(* Logix 5000 AddOnInstructionDefinition export AOI_NTron_7026TX_v1_2; software revision 20.04 *)

TYPE UDT_NTRON_Switch_Common_v1 :   // Created to use UDT_NTRON_CIP_Switch_v1
STRUCT
   Generic_Inputs : UDT_NTRON_Switch_In_v0;   // assembly received from switch
   Output : DINT;   // assembly sent to switch
   Identity : UDT_NTRON_CIP_Identity_v0;
   TCPIP : UDT_NTRON_CIP_TCPIP_Interface_v0;
   Switch : UDT_NTRON_CIP_Switch_v1;
   Ethernet_Link : UDT_NTRON_CIP_Ethernet_Link_v0[64];
   Data : UDT_NTRON_CIP_DATA_v0;   // Related to HMI data and control
   Control : UDT_NTRON_CIP_Control_v0;
END_STRUCT
END_TYPE

TYPE UDT_NTRON_CIP_Interface_Control_v0 :
STRUCT
   Control_Bits : INT;
   Forced_Interface_Speed : INT;
END_STRUCT
END_TYPE

TYPE UDT_NTRON_Switch_7026TX_In_v0 :   // N-TRON 7026TX Switch 26 Port (24 10/100BaseTX, 2 SFP Mini-GBIC Gigabit Fiber Expansion Ports)
STRUCT
   System_Faults : UDT_NTRON_System_Faults_v0;
   Admin_Status : DINT;   // AdminStatus of first 32 ports
   Admin_Status_P1 : BOOL;   // 1=enabled, 0=disabled
   Admin_Status_P2 : BOOL;
   Admin_Status_P3 : BOOL;
   Admin_Status_P4 : BOOL;
   Admin_Status_P5 : BOOL;
   Admin_Status_P6 : BOOL;
   Admin_Status_P7 : BOOL;
   Admin_Status_P8 : BOOL;
   Admin_Status_P9 : BOOL;
   Admin_Status_P10 : BOOL;
   Admin_Status_P11 : BOOL;
   Admin_Status_P12 : BOOL;
   Admin_Status_P13 : BOOL;
   Admin_Status_P14 : BOOL;
   Admin_Status_P15 : BOOL;
   Admin_Status_P16 : BOOL;
   Admin_Status_P17 : BOOL;
   Admin_Status_P18 : BOOL;
   Admin_Status_P19 : BOOL;
   Admin_Status_P20 : BOOL;
   Admin_Status_P21 : BOOL;
   Admin_Status_P22 : BOOL;
   Admin_Status_P23 : BOOL;
   Admin_Status_P24 : BOOL;
   Admin_Status_P25 : BOOL;
   Admin_Status_P26 : BOOL;
   Link_Status : DINT;   // LinkStatus of first 32 ports
   Link_Status_P1 : BOOL;   // 1=active, 0=inactive
   Link_Status_P2 : BOOL;
   Link_Status_P3 : BOOL;
   Link_Status_P4 : BOOL;
   Link_Status_P5 : BOOL;
   Link_Status_P6 : BOOL;
   Link_Status_P7 : BOOL;
   Link_Status_P8 : BOOL;
   Link_Status_P9 : BOOL;
   Link_Status_P10 : BOOL;
   Link_Status_P11 : BOOL;
   Link_Status_P12 : BOOL;
   Link_Status_P13 : BOOL;
   Link_Status_P14 : BOOL;
   Link_Status_P15 : BOOL;
   Link_Status_P16 : BOOL;
   Link_Status_P17 : BOOL;
   Link_Status_P18 : BOOL;
   Link_Status_P19 : BOOL;
   Link_Status_P20 : BOOL;
   Link_Status_P21 : BOOL;
   Link_Status_P22 : BOOL;
   Link_Status_P23 : BOOL;
   Link_Status_P24 : BOOL;
   Link_Status_P25 : BOOL;
   Link_Status_P26 : BOOL;
   Utilization_Alarm : DINT;   // Bandwith utilization alarms for first 32 ports
   Utilization_Alarm_P1 : BOOL;
   Utilization_Alarm_P2 : BOOL;
   Utilization_Alarm_P3 : BOOL;
   Utilization_Alarm_P4 : BOOL;
   Utilization_Alarm_P5 : BOOL;
   Utilization_Alarm_P6 : BOOL;
   Utilization_Alarm_P7 : BOOL;
   Utilization_Alarm_P8 : BOOL;
   Utilization_Alarm_P9 : BOOL;
   Utilization_Alarm_P10 : BOOL;
   Utilization_Alarm_P11 : BOOL;
   Utilization_Alarm_P12 : BOOL;
   Utilization_Alarm_P13 : BOOL;
   Utilization_Alarm_P14 : BOOL;
   Utilization_Alarm_P15 : BOOL;
   Utilization_Alarm_P16 : BOOL;
   Utilization_Alarm_P17 : BOOL;
   Utilization_Alarm_P18 : BOOL;
   Utilization_Alarm_P19 : BOOL;
   Utilization_Alarm_P20 : BOOL;
   Utilization_Alarm_P21 : BOOL;
   Utilization_Alarm_P22 : BOOL;
   Utilization_Alarm_P23 : BOOL;
   Utilization_Alarm_P24 : BOOL;
   Utilization_Alarm_P25 : BOOL;
   Utilization_Alarm_P26 : BOOL;
   Class1_Connections : INT;   // Number of CIP Ethernet/IP class 1 (multicast) connections
   Class3_Connections : INT;   // Number of CIP Ethernet/IP class 3 (unicast) connections
   Temperature_C : INT;   // Temperature in degrees Celsius. 0x7FFF = Not supported on device.
   Temperature_F : INT;   // Temperature in degrees Fahrenheit. 0x7FFF = Not supported on device.
   CPU_Utilization : SINT;   // Percent of CPU usage, 0-100
   Contact_Status : SINT;   // 2 Bits per contact. 00=Not Present, 01=Open, 10=Closed.
   Utilization_P1 : SINT;
   Utilization_P2 : SINT;
   Utilization_P3 : SINT;
   Utilization_P4 : SINT;
   Utilization_P5 : SINT;
   Utilization_P6 : SINT;
   Utilization_P7 : SINT;
   Utilization_P8 : SINT;
   Utilization_P9 : SINT;
   Utilization_P10 : SINT;
   Utilization_P11 : SINT;
   Utilization_P12 : SINT;
   Utilization_P13 : SINT;
   Utilization_P14 : SINT;
   Utilization_P15 : SINT;
   Utilization_P16 : SINT;
   Utilization_P17 : SINT;
   Utilization_P18 : SINT;
   Utilization_P19 : SINT;
   Utilization_P20 : SINT;
   Utilization_P21 : SINT;
   Utilization_P22 : SINT;
   Utilization_P23 : SINT;
   Utilization_P24 : SINT;
   Utilization_P25 : SINT;
   Utilization_P26 : SINT;
END_STRUCT
END_TYPE

TYPE UDT_NTRON_CIP_DATA_v0 :   // This UDT contains various information that appears on an HMI display. Some information applies to the switch, and some applies to the selected port (copied, or derived from, the port Ethernet_Link data) because FactoryTalk can not access array elements.
STRUCT
   Switch_Name : STRING;
   IP_Address : UDT_NTRON_String32;
   Subnet_Mask : UDT_NTRON_String32;
   Gateway_Address : UDT_NTRON_String32;
   Port_Speed : DINT;   // begin port specific data
   Port_Interface_Flags : UDT_NTRON_CIP_Interface_Flags_v0;
   Port_Interface_Label : STRING;
   Port_Interface_Type : SINT;   // 0-unknown, 1-internal, 2-twisted pair, 3-optical
   InOctets : DINT;
   InUcastPackets : DINT;
   InNucastPackets : DINT;
   OutOctets : DINT;
   OutUcastPackets : DINT;
   OutNucastPackets : DINT;
   Port : SINT;   // end port specific data
   MAC_Address : UDT_NTRON_String32;   // MAC address of switch
   TX_Unicast_Packet_Rate : DINT;   // begin port specific data
   RX_Unicast_Packet_Rate : DINT;
   TX_Multicast_Packet_Rate : DINT;
   RX_Multicast_Packet_Rate : DINT;
   TX_Broadcast_Packet_Rate : DINT;
   RX_Broadcast_Packet_Rate : DINT;
   Interface_Utilization : SINT;
   Port_Role : DINT;
   Error_Count : DINT;
   Fault_Count : DINT;   // end port specific data
   AOI_Major_Version : DINT;   // The faceplate reads this version to determine if the AOI tags can be used by the faceplate. If not, a warning is displayed.
   AOI_Minor_Version : DINT;   // The faceplate reads this version to determine if the AOI tags can be used by the faceplate. If not, a warning is displayed.
   CIP_Version_Fault : BOOL;   // True if the switch CIP version does not support this version of the AOI, otherwise false.
   Stale_Data : BOOL;   // True if assembly data has not been received lately.
   System_Fault_String : UDT_NTRON_String480;
END_STRUCT
END_TYPE

TYPE UDT_NTRON_CIP_Interface_Flags_v0 :
STRUCT
   Link_Status : BOOL;   // 0-inactive, 1-active
   Duplex : BOOL;   // 0-half, 1-full
   Negotiation_Status_1 : BOOL;
   Negotiation_Status_2 : BOOL;
   Negotiation_Status_3 : BOOL;
   Manual_Setting_Requires_Reset : BOOL;
   Local_Hardware_Fault : BOOL;
END_STRUCT
END_TYPE

TYPE UDT_NTRON_CIP_Control_v0 :   // Created to control explicit CIP messaging
STRUCT
   HMI : UDT_NTRON_HMI_Control_v0[1];   // Read Ethernet Link object for the selected port. 0=disabled.
   Selected_Port : INT;   // Use this member to read Ethernet Link object for one port. To read more than one port, use Read_Port_Mask. Set by the faceplate. Port data is copied to the UDT_NTRON_CIP_DATA_v0 data type.
   Request_Data : BOOL;   // 0 - explicit messaging is disabled; 1 - explicit messaging is enabled
   Read_Port_Mask : DINT;   // Set bit n to read ethernet link object for port n+1
   Read_Port_Mask2 : DINT;   // Set bit n to read ethernet link object for port n+33
   Explicit_Messaging_Timer_Reset : DINT;   // Used to control time between each MSG call to read CIP Identity object, TCPIP object, N-TRON object, and selected Ethernet Link objects. Minimum is 200 ms. Default is 1000 ms.
END_STRUCT
END_TYPE

TYPE UDT_NTRON_CIP_TCPIP_Interface_v0 :   // N-TRON CIP TCP/IP Interface Object
STRUCT
   Status : DINT;   // Interface status
   Configuration_Capability : DINT;   // Interface capability flags
   Configuration_Control : DINT;   // Interface control flags
   Path_Size : INT;   // Size of Path
   Object_Path_1 : INT;   // Logical segments identifying the physical link object
   Object_Path_2 : INT;   // Logical segments identifying the physical link object
   IP_Address : DINT;   // The device’s IP address.
   Network_Mask : DINT;   // The device’s network mask
   Gateway_Address : DINT;   // Default gateway address
   Name_Server_1 : DINT;   // Primary name server
   Name_Server_2 : DINT;   // Secondary name server
   Domain_Name : STRING;   // Default domain name
   Host_Name : STRING;   // Host name
END_STRUCT
END_TYPE

TYPE UDT_NTRON_Switch_In_v0 :   // Generic view of assembly data received from an N-TRON Switch. This UDT must match exactly the assembly sent from the switch.
STRUCT
   System_Faults : UDT_NTRON_System_Faults_v0;   // Status of various system faults.
   Admin_Status : DINT;   // Admin_Status of first 32 ports. Also available as port specific tags.
   Admin_Status_1 : BOOL;   // 1=enabled, 0=disabled
   Admin_Status_2 : BOOL;
   Admin_Status_3 : BOOL;
   Admin_Status_4 : BOOL;
   Admin_Status_5 : BOOL;
   Admin_Status_6 : BOOL;
   Admin_Status_7 : BOOL;
   Admin_Status_8 : BOOL;
   Admin_Status_9 : BOOL;
   Admin_Status_10 : BOOL;
   Admin_Status_11 : BOOL;
   Admin_Status_12 : BOOL;
   Admin_Status_13 : BOOL;
   Admin_Status_14 : BOOL;
   Admin_Status_15 : BOOL;
   Admin_Status_16 : BOOL;
   Admin_Status_17 : BOOL;
   Admin_Status_18 : BOOL;
   Admin_Status_19 : BOOL;
   Admin_Status_20 : BOOL;
   Admin_Status_21 : BOOL;
   Admin_Status_22 : BOOL;
   Admin_Status_23 : BOOL;
   Admin_Status_24 : BOOL;
   Admin_Status_25 : BOOL;
   Admin_Status_26 : BOOL;
   Admin_Status_27 : BOOL;
   Admin_Status_28 : BOOL;
   Admin_Status_29 : BOOL;
   Admin_Status_30 : BOOL;
   Admin_Status_31 : BOOL;
   Admin_Status_32 : BOOL;
   Admin_Status2 : DINT;   // Admin_Status of second 32 ports. Also available as port specific tags.
   Admin_Status_33 : BOOL;   // 1=enabled, 0=disabled
   Admin_Status_34 : BOOL;
   Admin_Status_35 : BOOL;
   Admin_Status_36 : BOOL;
   Admin_Status_37 : BOOL;
   Admin_Status_38 : BOOL;
   Admin_Status_39 : BOOL;
   Admin_Status_40 : BOOL;
   Admin_Status_41 : BOOL;
   Admin_Status_42 : BOOL;
   Admin_Status_43 : BOOL;
   Admin_Status_44 : BOOL;
   Admin_Status_45 : BOOL;
   Admin_Status_46 : BOOL;
   Admin_Status_47 : BOOL;
   Admin_Status_48 : BOOL;
   Admin_Status_49 : BOOL;
   Admin_Status_50 : BOOL;
   Admin_Status_51 : BOOL;
   Admin_Status_52 : BOOL;
   Admin_Status_53 : BOOL;
   Admin_Status_54 : BOOL;
   Admin_Status_55 : BOOL;
   Admin_Status_56 : BOOL;
   Admin_Status_57 : BOOL;
   Admin_Status_58 : BOOL;
   Admin_Status_59 : BOOL;
   Admin_Status_60 : BOOL;
   Admin_Status_61 : BOOL;
   Admin_Status_62 : BOOL;
   Admin_Status_63 : BOOL;
   Admin_Status_64 : BOOL;
   Link_Status : DINT;   // Link_Status of first 32 ports. Also available as port specific tags.
   Link_Status_1 : BOOL;   // 1=active, 0=inactive
   Link_Status_2 : BOOL;
   Link_Status_3 : BOOL;
   Link_Status_4 : BOOL;
   Link_Status_5 : BOOL;
   Link_Status_6 : BOOL;
   Link_Status_7 : BOOL;
   Link_Status_8 : BOOL;
   Link_Status_9 : BOOL;
   Link_Status_10 : BOOL;
   Link_Status_11 : BOOL;
   Link_Status_12 : BOOL;
   Link_Status_13 : BOOL;
   Link_Status_14 : BOOL;
   Link_Status_15 : BOOL;
   Link_Status_16 : BOOL;
   Link_Status_17 : BOOL;
   Link_Status_18 : BOOL;
   Link_Status_19 : BOOL;
   Link_Status_20 : BOOL;
   Link_Status_21 : BOOL;
   Link_Status_22 : BOOL;
   Link_Status_23 : BOOL;
   Link_Status_24 : BOOL;
   Link_Status_25 : BOOL;
   Link_Status_26 : BOOL;
   Link_Status_27 : BOOL;
   Link_Status_28 : BOOL;
   Link_Status_29 : BOOL;
   Link_Status_30 : BOOL;
   Link_Status_31 : BOOL;
   Link_Status_32 : BOOL;
   Link_Status2 : DINT;   // Link_Status of second 32 ports. Also available as port specific tags.
   Link_Status_33 : BOOL;   // 1=active, 0=inactive
   Link_Status_34 : BOOL;
   Link_Status_35 : BOOL;
   Link_Status_36 : BOOL;
   Link_Status_37 : BOOL;
   Link_Status_38 : BOOL;
   Link_Status_39 : BOOL;
   Link_Status_40 : BOOL;
   Link_Status_41 : BOOL;
   Link_Status_42 : BOOL;
   Link_Status_43 : BOOL;
   Link_Status_44 : BOOL;
   Link_Status_45 : BOOL;
   Link_Status_46 : BOOL;
   Link_Status_47 : BOOL;
   Link_Status_48 : BOOL;
   Link_Status_49 : BOOL;
   Link_Status_50 : BOOL;
   Link_Status_51 : BOOL;
   Link_Status_52 : BOOL;
   Link_Status_53 : BOOL;
   Link_Status_54 : BOOL;
   Link_Status_55 : BOOL;
   Link_Status_56 : BOOL;
   Link_Status_57 : BOOL;
   Link_Status_58 : BOOL;
   Link_Status_59 : BOOL;
   Link_Status_60 : BOOL;
   Link_Status_61 : BOOL;
   Link_Status_62 : BOOL;
   Link_Status_63 : BOOL;
   Link_Status_64 : BOOL;
   Utilization_Alarm : DINT;   // Bandwith utilization alarms for first 32 ports. Also available as port specific tags.
   Utilization_Alarm_1 : BOOL;   // 1=bandwidth utilization exceeds a high or low limit, 0=bandwidth utilization within limits
   Utilization_Alarm_2 : BOOL;
   Utilization_Alarm_3 : BOOL;
   Utilization_Alarm_4 : BOOL;
   Utilization_Alarm_5 : BOOL;
   Utilization_Alarm_6 : BOOL;
   Utilization_Alarm_7 : BOOL;
   Utilization_Alarm_8 : BOOL;
   Utilization_Alarm_9 : BOOL;
   Utilization_Alarm_10 : BOOL;
   Utilization_Alarm_11 : BOOL;
   Utilization_Alarm_12 : BOOL;
   Utilization_Alarm_13 : BOOL;
   Utilization_Alarm_14 : BOOL;
   Utilization_Alarm_15 : BOOL;
   Utilization_Alarm_16 : BOOL;
   Utilization_Alarm_17 : BOOL;
   Utilization_Alarm_18 : BOOL;
   Utilization_Alarm_19 : BOOL;
   Utilization_Alarm_20 : BOOL;
   Utilization_Alarm_21 : BOOL;
   Utilization_Alarm_22 : BOOL;
   Utilization_Alarm_23 : BOOL;
   Utilization_Alarm_24 : BOOL;
   Utilization_Alarm_25 : BOOL;
   Utilization_Alarm_26 : BOOL;
   Utilization_Alarm_27 : BOOL;
   Utilization_Alarm_28 : BOOL;
   Utilization_Alarm_29 : BOOL;
   Utilization_Alarm_30 : BOOL;
   Utilization_Alarm_31 : BOOL;
   Utilization_Alarm_32 : BOOL;
   Utilization_Alarm2 : DINT;   // Bandwith utilization alarms for second 32 ports. Also available as port specific tags.
   Utilization_Alarm_33 : BOOL;   // 1=bandwidth utilization exceeds a high or low limit, 0=bandwidth utilization within limits
   Utilization_Alarm_34 : BOOL;
   Utilization_Alarm_35 : BOOL;
   Utilization_Alarm_36 : BOOL;
   Utilization_Alarm_37 : BOOL;
   Utilization_Alarm_38 : BOOL;
   Utilization_Alarm_39 : BOOL;
   Utilization_Alarm_40 : BOOL;
   Utilization_Alarm_41 : BOOL;
   Utilization_Alarm_42 : BOOL;
   Utilization_Alarm_43 : BOOL;
   Utilization_Alarm_44 : BOOL;
   Utilization_Alarm_45 : BOOL;
   Utilization_Alarm_46 : BOOL;
   Utilization_Alarm_47 : BOOL;
   Utilization_Alarm_48 : BOOL;
   Utilization_Alarm_49 : BOOL;
   Utilization_Alarm_50 : BOOL;
   Utilization_Alarm_51 : BOOL;
   Utilization_Alarm_52 : BOOL;
   Utilization_Alarm_53 : BOOL;
   Utilization_Alarm_54 : BOOL;
   Utilization_Alarm_55 : BOOL;
   Utilization_Alarm_56 : BOOL;
   Utilization_Alarm_57 : BOOL;
   Utilization_Alarm_58 : BOOL;
   Utilization_Alarm_59 : BOOL;
   Utilization_Alarm_60 : BOOL;
   Utilization_Alarm_61 : BOOL;
   Utilization_Alarm_62 : BOOL;
   Utilization_Alarm_63 : BOOL;
   Utilization_Alarm_64 : BOOL;
   Class1_Connections : INT;   // Number of CIP Ethernet/IP class 1 (multicast) connections
   Class3_Connections : INT;   // Number of CIP Ethernet/IP class 3 (unicast) connections
   Temperature_C : INT;   // Temperature in degrees Celsius. 0x7FFF = Not supported on device.
   Temperature_F : INT;   // Temperature in degrees Fahrenheit. 0x7FFF = Not supported on device.
   CPU_Utilization : SINT;   // Percent of CPU usage, 0-100
   Contact_Status : SINT;   // 2 Bits per contact. 00=Not Present, 01=Open, 10=Closed.
   Utilization_1 : SINT;   // bandwidth utilization in percent
   Utilization_2 : SINT;
   Utilization_3 : SINT;
   Utilization_4 : SINT;
   Utilization_5 : SINT;
   Utilization_6 : SINT;
   Utilization_7 : SINT;
   Utilization_8 : SINT;
   Utilization_9 : SINT;
   Utilization_10 : SINT;
   Utilization_11 : SINT;
   Utilization_12 : SINT;
   Utilization_13 : SINT;
   Utilization_14 : SINT;
   Utilization_15 : SINT;
   Utilization_16 : SINT;
   Utilization_17 : SINT;
   Utilization_18 : SINT;
   Utilization_19 : SINT;
   Utilization_20 : SINT;
   Utilization_21 : SINT;
   Utilization_22 : SINT;
   Utilization_23 : SINT;
   Utilization_24 : SINT;
   Utilization_25 : SINT;
   Utilization_26 : SINT;
   Utilization_27 : SINT;
   Utilization_28 : SINT;
   Utilization_29 : SINT;
   Utilization_30 : SINT;
   Utilization_31 : SINT;
   Utilization_32 : SINT;
   Utilization_33 : SINT;
   Utilization_34 : SINT;
   Utilization_35 : SINT;
   Utilization_36 : SINT;
   Utilization_37 : SINT;
   Utilization_38 : SINT;
   Utilization_39 : SINT;
   Utilization_40 : SINT;
   Utilization_41 : SINT;
   Utilization_42 : SINT;
   Utilization_43 : SINT;
   Utilization_44 : SINT;
   Utilization_45 : SINT;
   Utilization_46 : SINT;
   Utilization_47 : SINT;
   Utilization_48 : SINT;
   Utilization_49 : SINT;
   Utilization_50 : SINT;
   Utilization_51 : SINT;
   Utilization_52 : SINT;
   Utilization_53 : SINT;
   Utilization_54 : SINT;
   Utilization_55 : SINT;
   Utilization_56 : SINT;
   Utilization_57 : SINT;
   Utilization_58 : SINT;
   Utilization_59 : SINT;
   Utilization_60 : SINT;
   Utilization_61 : SINT;
   Utilization_62 : SINT;
   Utilization_63 : SINT;
   Utilization_64 : SINT;
   Update_Counter : INT;
END_STRUCT
END_TYPE

TYPE UDT_NTRON_System_Faults_v0 :   // Fault bits.
STRUCT
   Faults : DINT;
   Power_Supply_1 : BOOL;   // 1=Indicates a low voltage on power supply V1
   Power_Supply_2 : BOOL;   // 1=Indicates a low voltage on power supply V2
   NRing_Full : BOOL;   // 1=Indicates that an N-Ring connection is completely broken.
   NRing_Part_Low : BOOL;   // 1=Indicates that an N-Ring connection is only broken in one direction. The lower N-Ring port is not receiving self health frames around the N-Ring but the higher N-Ring port is.
   NRing_Part_High : BOOL;   // 1=Indicates that an N-Ring connection is only broken in one direction. The higher N-Ring port is not receiving self health frames around the N-Ring but the lower N-Ring port is.
   NRing_Multiple_Managers : BOOL;   // 1=Indicates that more than one N-Ring Manager exists on an N-Ring.
   System : BOOL;   // 1=Indicates a system fault.
   Config_Device : BOOL;   // 1=Indicates a problem with the configuration device.
   NLink : BOOL;   // 1=Indicates that the N-Link Master or Slave encountered a problem.
   Boot_Loader_Version : BOOL;   // 1=Indicates a problem with the version of the boot loader firmware.
   Port_Utilization : BOOL;   // 1=Indicates one or more ports have exceeded a high or low bandwidth utilization limit.
   Temperature : BOOL;   // 1=Indicates the switch temperature has exceeded a high or low temperature limit.
END_STRUCT
END_TYPE

TYPE UDT_NTRON_HMI_Set_v0 :   // Variables set by an HMI station. AOI sends changes to the switch. This UDT is used in combination with N-TRON's faceplates for FactoryTalk View.
STRUCT
   Speed_Duplex : SINT;   // 100=auto negotiate, 1=10/half, 2=10/full, 3=100/half, 4=100/full, 5=1000/half, 6=1000/full (Supported speed/duplex combinations are switch dependent.)
   Admin_Enable : SINT;   // 1=enable, 2=disable
   Enter_Speed_Duplex : BOOL;   // Set to 1 to trigger speed/duplex change
   Enter_Admin_Enable : BOOL;   // Set to 1 to trigger admin enable/disable change
END_STRUCT
END_TYPE

TYPE UDT_NTRON_CIP_Identity_v0 :   // N-TRON CIP Identity Object
STRUCT
   Vendor_ID : INT;   // ODVA Vendor ID. N-Tron = 1006
   Device_Type : INT;   // 0x0C. Communications Adapter
   Product_Code : INT;   // 708TX=701, 708FX2=703, 716TX=705, 716FX2=706, 7018TX=708, 7018FX2=709, 708M12=710, 711FX3=711, 7010TX=713, 709FX=714, 710FX2=715, 714FX6=717, 712FX4=718, 7012FX2=719, 7026TX=720, 7506GX2=7506, 7900=722, 716M12=723
   Major_Revision : SINT;   // Major revision of the item the Identity Object represents
   Minor_Revision : SINT;   // Minor revision of the item the Identity Object represents
   Status : INT;   // Summary status of device
   Serial_Number : DINT;   // Serial number of device
   Product_Name : STRING;   // Human readable identification. Switch model number. Ex: N-TRON 7018FX2
   Assigned_Name : UDT_NTRON_String1024;   // User assigned switch name.
   Geographic_Location : UDT_NTRON_String1024;   // This is the user assigned switch location.
END_STRUCT
END_TYPE

TYPE UDT_NTRON_String32 :   // string type
STRUCT
   LEN : DINT;
   DATA : SINT[32];
END_STRUCT
END_TYPE

TYPE UDT_NTRON_HMI_Control_v0 :   // Settings written by HMI station. This UDT is used in combination with N-TRON's faceplates for FactoryTalk View.
STRUCT
   Selected_Port : INT;   // Current port selected on the FactoryTalk faceplate. 1=port 1, 2=port 2, etc.
   Set : UDT_NTRON_HMI_Set_v0;
   Display_Mode : SINT;   // Active Faceplate pane. 0=none, 1=main, 2=diagnostics, 3=settings, etc.
END_STRUCT
END_TYPE

TYPE UDT_NTRON_String1024 :   // string type
STRUCT
   LEN : DINT;
   DATA : SINT[1024];
END_STRUCT
END_TYPE

TYPE UDT_NTRON_String480 :   // string type; The "Maximum Characters" of this string type is based on the maximum length you can display in FactoryTalk View.
STRUCT
   LEN : DINT;
   DATA : SINT[480];
END_STRUCT
END_TYPE

TYPE UDT_NTRON_CIP_Ethernet_Link_v0 :   // N-TRON CIP Ethernet Link Object
STRUCT
   Interface_Speed : DINT;   // Interface speed currently in use. Speed in Mbps (e.g., 0, 10, 100, 1000, etc.)
   Interface_Flags : UDT_NTRON_CIP_Interface_Flags_v0;   // Interface status flags
   Physical_Address : SINT[6];   // MAC layer address
   InOctets : DINT;   // Octets received on the interface
   InUcastPackets : DINT;   // Unicast packets received on the interface
   InNucastPackets : DINT;   // Non-unicast packets received on the interface
   InDiscards : DINT;   // Inbound packets received on the interface but discarded
   InErrors : DINT;   // Inbound packets that contain errors (does not include In Discards)
   InUnknownProtos : DINT;   // Inbound packets with unknown protocol
   OutOctets : DINT;   // Octets sent on the interface
   OutUcastPackets : DINT;   // Unicast packets sent on the interface
   OutNucastPackets : DINT;   // Non-unicast packets sent on the interface
   OutDiscards : DINT;   // Outbound packets discarded
   OutErrors : DINT;   // Outbound packets that contain errors
   Alignment_Errors : DINT;   // Frames received that are not an integral number of octets in length
   FCS_Errors : DINT;   // Frames received that do not pass the FCS check
   Single_Collisions : DINT;   // Successfully transmitted frames which experienced exactly one collision
   Multiple_Collisions : DINT;   // Successfully transmitted frames which experienced more than one collision
   SQE_Test_Errors : DINT;   // Number of times SQE test error message is generated
   Deferred_Transmissions : DINT;   // Frames for which first transmission attempt is delayed because the medium is busy
   Late_Collisions : DINT;   // Number of times a collision is detected later than 512 bit- times into the transmission of a packet
   Excessive_Collisions : DINT;   // Frames for which transmission fails due to excessive collisions
   MAC_Transmit_Errors : DINT;   // Frames for which transmission fails due to an internal MAC sublayer transmit error
   Carrier_Sense_Errors : DINT;   // Times that the carrier sense condition was lost or never asserted when attempting to transmit a frame
   Frame_Too_Long : DINT;   // Frames received that exceed the maximum permitted frame size
   MAC_Receive_Errors : DINT;   // Frames for which reception on an interface fails due to an internal MAC sublayer receive error
   Control_Bits : INT;   // 0 Auto-negotiate 0 indicates 802.3 link auto-negotiation is disabled. 1 indicates auto-negotiation is enabled. If auto-negotiation is disabled, then the device shall use the settings indicated by the Forced Duplex Mode and Forced Interface Speed bits;. 1 Forced Duplex Mode If the Auto-negotiate bit is 0, the Forced Duplex Mode bit indicates whether the interface shall operate in full or half duplex mode. 0 indicates the interface duplex should be half duplex. 1 indicates the interface duplex
   Forced_Interface_Speed : INT;   // Speed at which the interface shall be forced to operate. Speed in Mbps (10, 100, 1000, etc.)
   Interface_Type : SINT;   // 0-unknown, 1-internal, 2-twisted pair, 3-optical
   Interface_State : SINT;   // 0-unknown, 1-enabled and ready, 2-disabled, 3-testing
   Admin_State : SINT;   // 1=enabled, 0=disabled
   Interface_Label : STRING;   // Label like "TX5"
   Interface_Description : STRING;   // Something like: Port 1 - 10/100 Mbit TX Port 15 - 100 MBit FX
   Interface_Utilization : SINT;   // Percentage of entire interface bandwidth being used (0-100)
   Utilization_Alarm_Upper_Threshold : SINT;   // Upper percentage at which to declare a utilization alarm (0-100).
   Utilization_Alarm_Lower_Threshold : SINT;   // Lower percentage at which to declare a utilization alarm (0-100).
   Broadcast_Limit : SINT;   // Broadcast limiting percentage (0-100). (BPCL)
   TX_Unicast_Packet_Rate : DINT;   // Number of TX unicast packets per second.
   RX_Unicast_Packet_Rate : DINT;   // Number of RX unicast packets per second.
   TX_Multicast_Packet_Rate : DINT;   // Number of TX multicast packets per second
   RX_Multicast_Packet_Rate : DINT;   // Number of RX multicast packets per second
   TX_Broadcast_Packet_Rate : DINT;   // Number of TX broadcast packets per second.
   RX_Broadcast_Packet_Rate : DINT;   // Number of RX broadcast packets per second
   TX_Multicast_Packets : DINT;   // Total number of TX multicast packets.
   RX_Multicast_Packets : DINT;   // Total number of RX multicast packets.
   TX_Broadcast_Packets : DINT;   // Total number of TX broadcast packets.
   RX_Broadcast_Packets : DINT;   // Total number of RX broadcast packets.
   Port_Role : DINT;   // Bit 0 = RSTP 1 = N-Ring 2 = N-Link Control 3 = N-Link Partner 4 = N-Link Coupler
END_STRUCT
END_TYPE

TYPE UDT_NTRON_CIP_Switch_v1 :   // N-TRON CIP Custom Object
STRUCT
   Device_Uptime : DINT;   // Number of seconds since device was powered up.
   Port_Count : DINT;   // Total port count
   Valid_Ports : DINT[2];   // 0 = Invalid port, 1 = Port exists on device Bit 0: Port 1 Bit 1: Port 2 etc.
   Global_Admin_Status : DINT[2];   // 0 = Port disabled, 1 = Port enabled Bit n: Port n+1
   Global_Link_Status : DINT[2];   // 0 = Link down, 1 = Link up Bit n: Port n+1
   System_Faults : UDT_NTRON_System_Faults_v0;   // Bit 00: Power Supply 1 Bit 01: Power Supply 2 Bit 02: N-Ring Fault (complete) Bit 03: N-Ring Partial Fault (low port) Bit 04: N-Ring Partial Fault (high port) Bit 05: N-Ring Multiple Managers Bit 06: System error Bit 07: Dongle Configuration Invalid Bit 08: N-Link Fault Bit 09: Boot loader version mismatch Bit 10: Port Utilization Alarm Bit 11: Temperature Alarm
   IGMP_Querier_Status : SINT;   // Query Status: 0 = Disabled, 1 = Active (manual), 2 = Active (Auto), 3 = Backup (Auto) [enabled but not active].
   IGMP_Version : SINT;   // IGMP Version (V1, V2, V3, etc).
   IGMP_Resource_Usage : SINT;   // Percent of maximum capacity. Takes into account the number of groups used per max groups and any other possible resource limitations.
   IGMP_Active_Querier : DINT;   // IP of the active IGMP querier.
   CPU_Usage : SINT;   // Percent usage
   Class1_Connections : INT;   // Number of CIP Ethernet/IP class 1 (multicast) connections.
   Class3_Connections : INT;   // Number of CIP Ethernet/IP class 3 (unicast) connections.
   Temperature_Alarm_Upper_Threshold : INT;   // Upper temperature (C) at which to declare an alarm
   Temperature_Alarm_Lower_Threshold : INT;   // Lower temperature (C) at which to declare an alarm
   Contact_Status : SINT;   // 2 Bits per contact. 00=Not Present, 01=Open, 10=Closed.
   Temperature_C : INT;   // Temperature in degrees C. Only available on devices that support temperature.
   Temperature_F : INT;   // Temperature in degrees F. Only available on devices that support temperature.
   Reset_MIB_Counts : DINT[2];   // Reset port MIB counters. (1 bit per port to reset).
   Device_MAC_Address : SINT[6];   // MAC address of device
   Device_Role : DINT;   // Bit mask of device roles. Bits= 0 = N-Ring Manager 1 = N-Ring Member 2 = N-Ring AutoDetect 3 = N-Link Master 4 = N-Link Slave 5 = N-Link Coupler
   Config_Device_Status : SINT;   // 0 = Not Supported, 1 = Not Present, 2 = Present
   System_Configuration : DINT;   // Bit mask of system config. Bits= 0 = Save system configuration to flash 1 = Shutdown and reboot device
   System_Firmware_Version_String : STRING;   // Human readable representation of firmware version string.
   System_Boot_Loader_Version_String : STRING;   // Human readable representation of boot loader version string.
   System_Fault_String : UDT_NTRON_String1024;   // Human readable representation of error status. May contain multiple errors. Length is contained as part of the STRINGI data type.
   Power_Configuration : DINT;   // 4 Bits per power supply. 0000 = DC Power (10-30 VDC) , 0001 = AC Power
   Miscellaneous_Status : DINT;   // Reserved for miscellaneous status
END_STRUCT
END_TYPE

ADD_ON_INSTRUCTION AOI_NTron_CIP_STRINGI_Copy_v1_0   (* revision 1.0, vendor Red Lion Controls, Inc. *)
// Copy a string formatted as a CIP STRINGI  to a UDT_NTRON_String1024 string.
// (C) 2015 Red Lion Controls, Inc. All rights reserved.
VAR_IN_OUT
   Input : SINT[1034]; {required}
   Output : UDT_NTRON_String1024; {required}
   indexInOut : DINT; {required}
END_VAR
VAR
   kStringI_ShortString : SINT := 16#da;   // Indicates a short string, which has the string length in one byte
   kStringI_String : SINT := 16#d0;   // Indicates a short string, which has the string length in two bytes
   index : DINT;
END_VAR

ROUTINE Logic   (* ladder *)
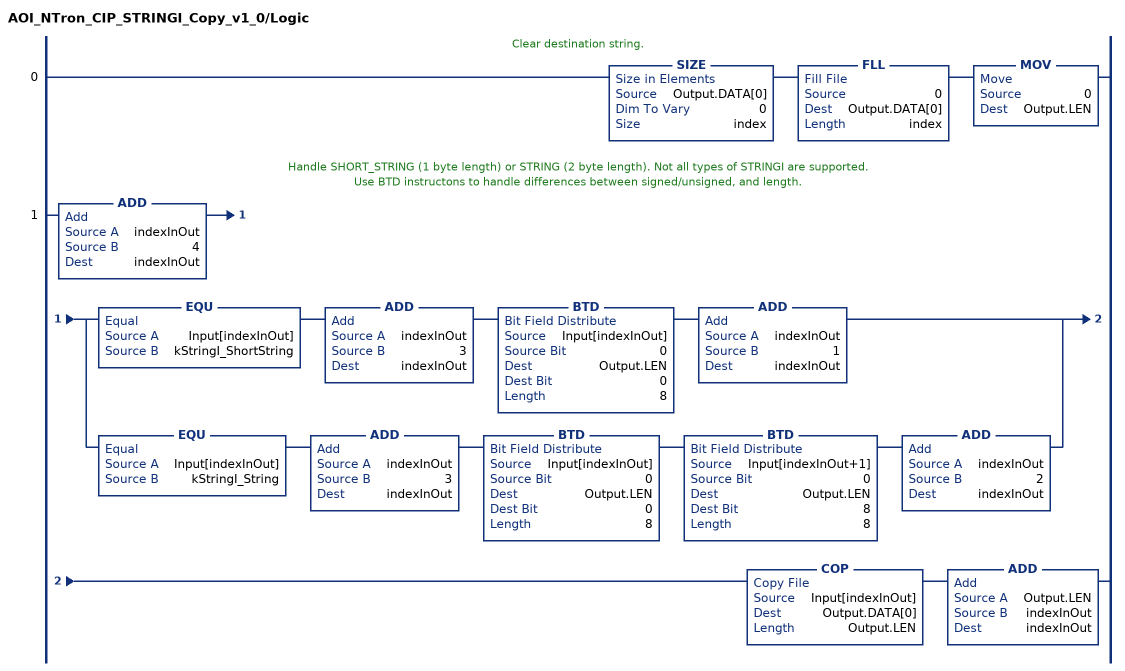
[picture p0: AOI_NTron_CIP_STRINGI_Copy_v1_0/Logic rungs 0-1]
   // Clear destination string.
   0: SIZE(Output.DATA[0],0,index)FLL(0,Output.DATA[0],index)MOV(0,Output.LEN);
   // Handle SHORT_STRING (1 byte length) or STRING (2 byte length). Not all types of STRINGI are supported.
   // Use BTD instructons to handle differences between signed/unsigned, and length.
   1: ADD(indexInOut,4,indexInOut)[EQU(Input[indexInOut],kStringI_ShortString) ADD(indexInOut,3,indexInOut) BTD(Input[indexInOut],0,Output.LEN,0,8) ADD(indexInOut,1,indexInOut) ,EQU(Input[indexInOut],kStringI_String) ADD(indexInOut,3,indexInOut) BTD(Input[indexInOut],0,Output.LEN,0,8) BTD(Input[indexInOut+1],0,Output.LEN,8,8) ADD(indexInOut,2,indexInOut) ]COP(Input[indexInOut],Output.DATA[0],Output.LEN)ADD(Output.LEN,indexInOut,indexInOut);
END_ROUTINE
END_ADD_ON_INSTRUCTION

ADD_ON_INSTRUCTION AOI_NTron_IP_Address_to_String_v1_0   (* revision 1.0, vendor Rockwell Automation *)
// Converts IP address obtained from TCP/IP CIP object to user-readable string. This AOI was obtained from the Rockwell sample code website.
// Help:
// AOI to convert a numerical IP address into a string in dotted decimal format
// Enter input DINT containing IP address in Numerical IP address field.
// Enter STRING variable to contain output in Readable IP address field
VAR_IN_OUT
   Numerical_IP_Address : DINT; {required}
   Readable_IP_Address : UDT_NTRON_String32; {required}
END_VAR
VAR
   Octet : DINT[4];
   StrOctet : UDT_NTRON_String32[4];
   Dot : STRING;
   Old_IP : DINT;
   Bools : DINT;
        .0   // One Shot Bit
        .1   // New_IP
END_VAR

ROUTINE Logic   (* ladder *)
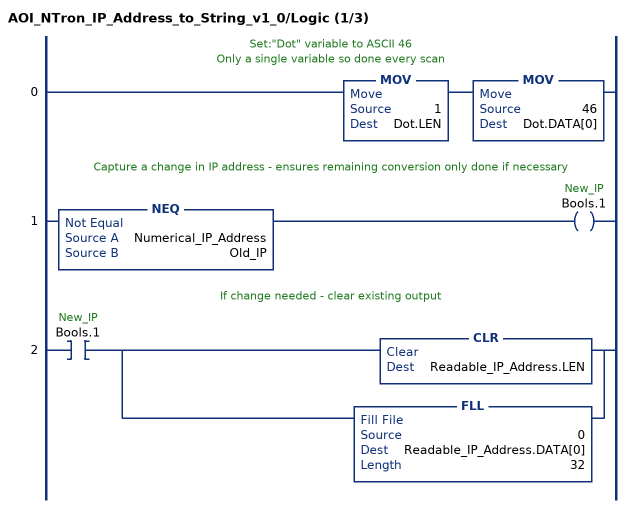
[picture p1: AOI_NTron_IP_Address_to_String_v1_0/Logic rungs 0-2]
   // Set:"Dot" variable to ASCII 46
   // Only a single variable so done every scan
   0: MOV(1,Dot.LEN)MOV(46,Dot.DATA[0]);
   // Capture a change in IP address - ensures remaining conversion only done if necessary
   1: NEQ(Numerical_IP_Address,Old_IP)OTE(Bools.1);
   // If change needed - clear existing output
   2: XIC(Bools.1)[CLR(Readable_IP_Address.LEN) ,FLL(0,Readable_IP_Address.DATA[0],32) ];
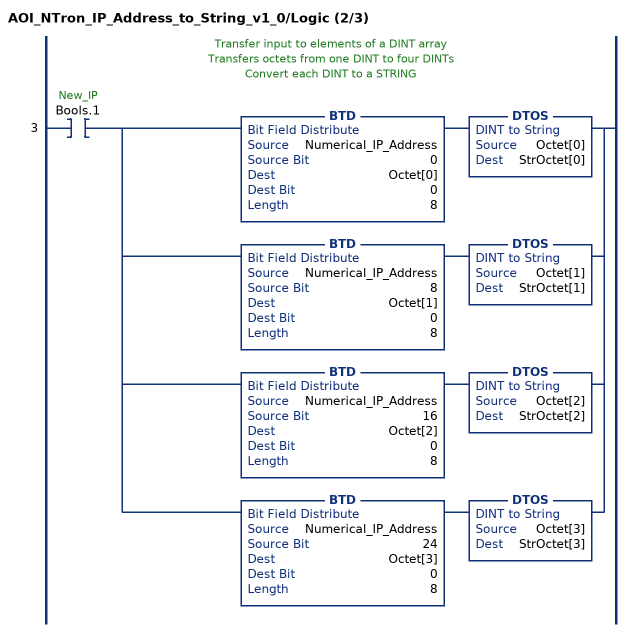
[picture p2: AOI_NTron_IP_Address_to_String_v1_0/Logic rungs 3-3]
   // Transfer input to elements of a DINT array
   // Transfers octets from one DINT to four DINTs
   // Convert each DINT to a STRING
   3: XIC(Bools.1)[BTD(Numerical_IP_Address,0,Octet[0],0,8) DTOS(Octet[0],StrOctet[0]) ,BTD(Numerical_IP_Address,8,Octet[1],0,8) DTOS(Octet[1],StrOctet[1]) ,BTD(Numerical_IP_Address,16,Octet[2],0,8) DTOS(Octet[2],StrOctet[2]) ,BTD(Numerical_IP_Address,24,Octet[3],0,8) DTOS(Octet[3],StrOctet[3]) ];
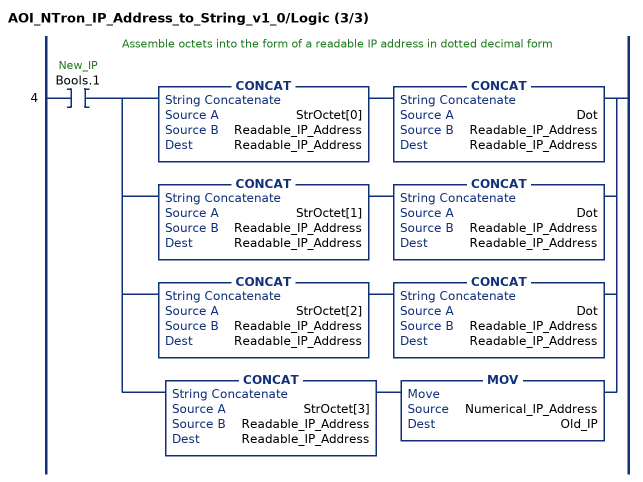
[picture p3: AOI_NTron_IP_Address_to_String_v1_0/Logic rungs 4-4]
   // Assemble octets into the form of a readable IP address in dotted decimal form
   4: XIC(Bools.1)[CONCAT(StrOctet[0],Readable_IP_Address,Readable_IP_Address) CONCAT(Dot,Readable_IP_Address,Readable_IP_Address) ,CONCAT(StrOctet[1],Readable_IP_Address,Readable_IP_Address) CONCAT(Dot,Readable_IP_Address,Readable_IP_Address) ,CONCAT(StrOctet[2],Readable_IP_Address,Readable_IP_Address) CONCAT(Dot,Readable_IP_Address,Readable_IP_Address) ,CONCAT(StrOctet[3],Readable_IP_Address,Readable_IP_Address) MOV(Numerical_IP_Address,Old_IP) ];
END_ROUTINE
END_ADD_ON_INSTRUCTION

ADD_ON_INSTRUCTION AOI_NTron_MAC_To_String_v1_0   (* revision 1.0, vendor Red Lion Controls, Inc. *)
// Convert MAC address to a string like 00.07.AF.FE.8F.A0.
// (C) 2015 Red Lion Controls, Inc. All rights reserved.
VAR_IN_OUT
   MAC : SINT[6]; {required}
   MAC_String : UDT_NTRON_String32; {required}
END_VAR
VAR
   nibble : SINT[12];
   index : SINT;
   nib : SINT;
END_VAR

ROUTINE Logic   (* ladder *)
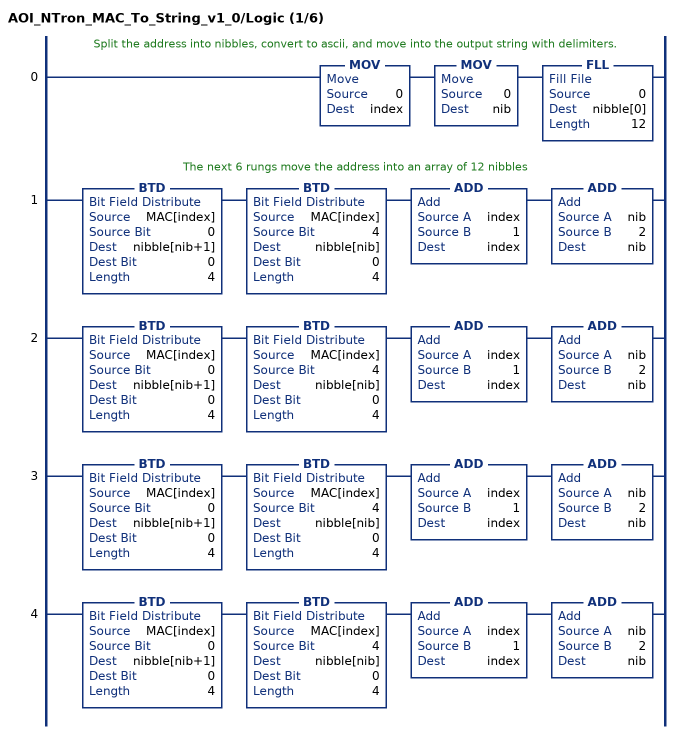
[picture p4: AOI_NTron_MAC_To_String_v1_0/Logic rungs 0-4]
   // Split the address into nibbles, convert to ascii, and move into the output string with delimiters.
   0: MOV(0,index)MOV(0,nib)FLL(0,nibble[0],12);
   // The next 6 rungs move the address into an array of 12 nibbles
   1: BTD(MAC[index],0,nibble[nib+1],0,4)BTD(MAC[index],4,nibble[nib],0,4)ADD(index,1,index)ADD(nib,2,nib);
   2: BTD(MAC[index],0,nibble[nib+1],0,4)BTD(MAC[index],4,nibble[nib],0,4)ADD(index,1,index)ADD(nib,2,nib);
   3: BTD(MAC[index],0,nibble[nib+1],0,4)BTD(MAC[index],4,nibble[nib],0,4)ADD(index,1,index)ADD(nib,2,nib);
   4: BTD(MAC[index],0,nibble[nib+1],0,4)BTD(MAC[index],4,nibble[nib],0,4)ADD(index,1,index)ADD(nib,2,nib);
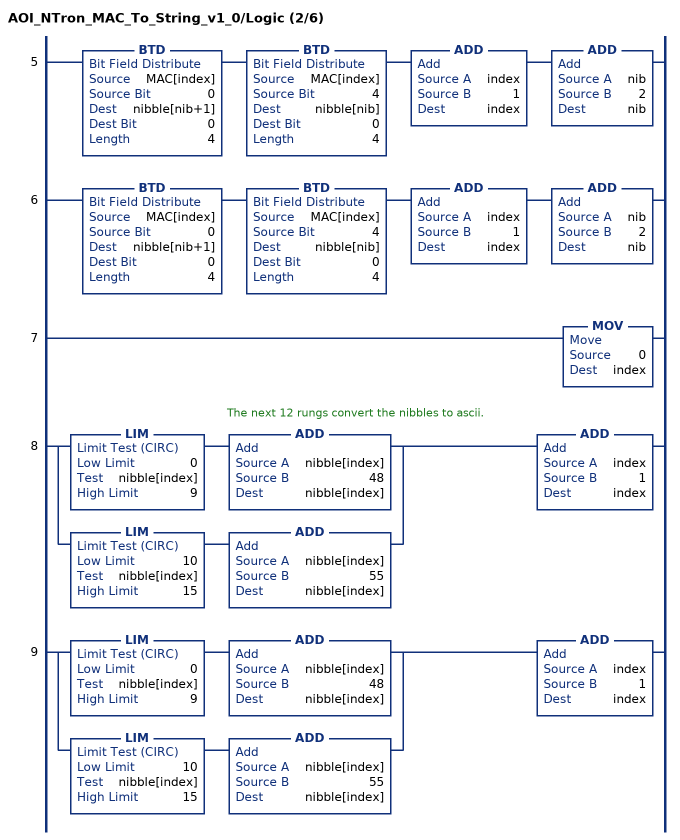
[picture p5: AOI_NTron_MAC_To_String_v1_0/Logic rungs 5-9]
   5: BTD(MAC[index],0,nibble[nib+1],0,4)BTD(MAC[index],4,nibble[nib],0,4)ADD(index,1,index)ADD(nib,2,nib);
   6: BTD(MAC[index],0,nibble[nib+1],0,4)BTD(MAC[index],4,nibble[nib],0,4)ADD(index,1,index)ADD(nib,2,nib);
   7: MOV(0,index);
   // The next 12 rungs convert the nibbles to ascii.
   8: [LIM(0,nibble[index],9) ADD(nibble[index],48,nibble[index]) ,LIM(10,nibble[index],15) ADD(nibble[index],55,nibble[index]) ]ADD(index,1,index);
   9: [LIM(0,nibble[index],9) ADD(nibble[index],48,nibble[index]) ,LIM(10,nibble[index],15) ADD(nibble[index],55,nibble[index]) ]ADD(index,1,index);
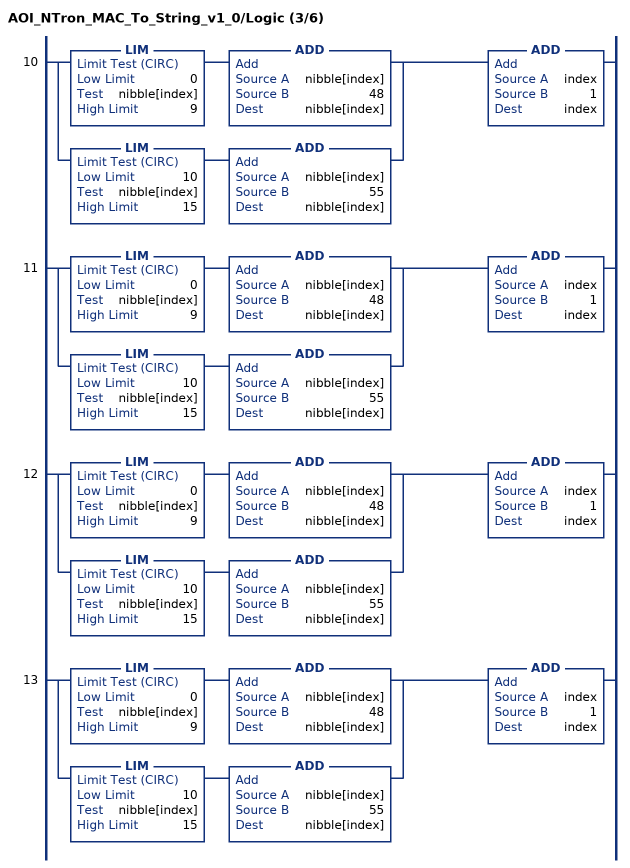
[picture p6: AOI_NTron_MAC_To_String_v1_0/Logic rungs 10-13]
   10: [LIM(0,nibble[index],9) ADD(nibble[index],48,nibble[index]) ,LIM(10,nibble[index],15) ADD(nibble[index],55,nibble[index]) ]ADD(index,1,index);
   11: [LIM(0,nibble[index],9) ADD(nibble[index],48,nibble[index]) ,LIM(10,nibble[index],15) ADD(nibble[index],55,nibble[index]) ]ADD(index,1,index);
   12: [LIM(0,nibble[index],9) ADD(nibble[index],48,nibble[index]) ,LIM(10,nibble[index],15) ADD(nibble[index],55,nibble[index]) ]ADD(index,1,index);
   13: [LIM(0,nibble[index],9) ADD(nibble[index],48,nibble[index]) ,LIM(10,nibble[index],15) ADD(nibble[index],55,nibble[index]) ]ADD(index,1,index);
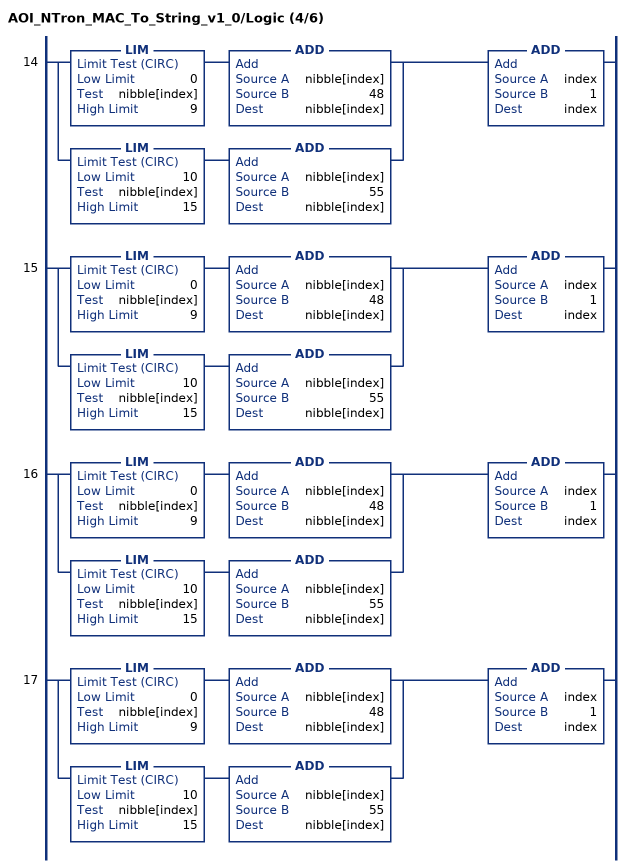
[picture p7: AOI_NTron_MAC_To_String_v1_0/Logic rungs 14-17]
   14: [LIM(0,nibble[index],9) ADD(nibble[index],48,nibble[index]) ,LIM(10,nibble[index],15) ADD(nibble[index],55,nibble[index]) ]ADD(index,1,index);
   15: [LIM(0,nibble[index],9) ADD(nibble[index],48,nibble[index]) ,LIM(10,nibble[index],15) ADD(nibble[index],55,nibble[index]) ]ADD(index,1,index);
   16: [LIM(0,nibble[index],9) ADD(nibble[index],48,nibble[index]) ,LIM(10,nibble[index],15) ADD(nibble[index],55,nibble[index]) ]ADD(index,1,index);
   17: [LIM(0,nibble[index],9) ADD(nibble[index],48,nibble[index]) ,LIM(10,nibble[index],15) ADD(nibble[index],55,nibble[index]) ]ADD(index,1,index);
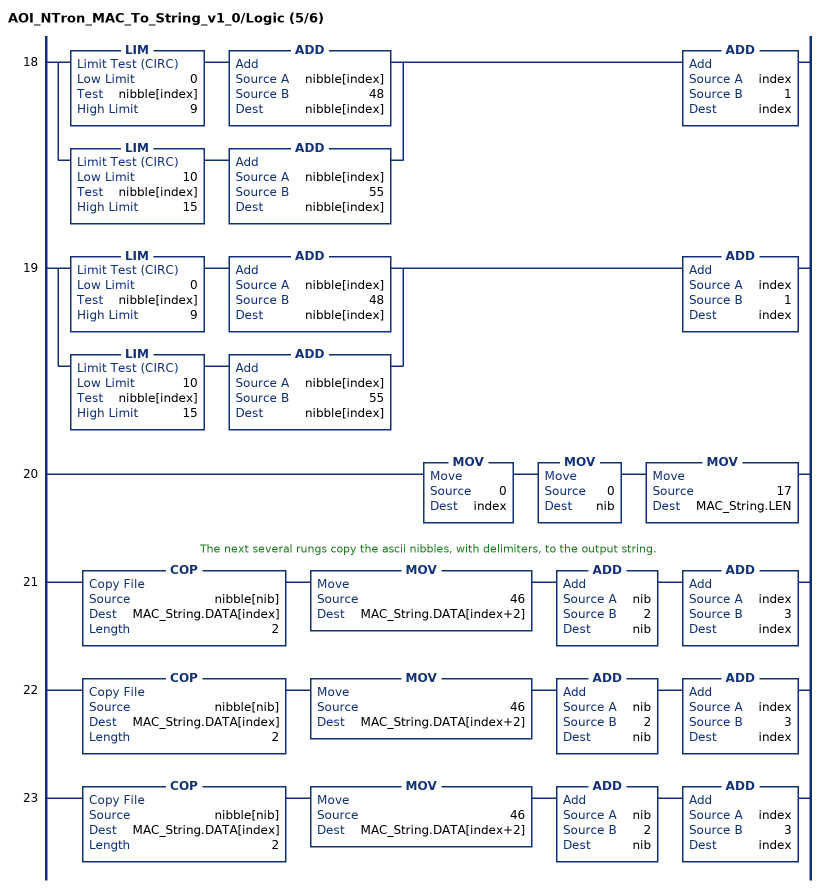
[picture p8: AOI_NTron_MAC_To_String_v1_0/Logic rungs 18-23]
   18: [LIM(0,nibble[index],9) ADD(nibble[index],48,nibble[index]) ,LIM(10,nibble[index],15) ADD(nibble[index],55,nibble[index]) ]ADD(index,1,index);
   19: [LIM(0,nibble[index],9) ADD(nibble[index],48,nibble[index]) ,LIM(10,nibble[index],15) ADD(nibble[index],55,nibble[index]) ]ADD(index,1,index);
   20: MOV(0,index)MOV(0,nib)MOV(17,MAC_String.LEN);
   // The next several rungs copy the ascii nibbles, with delimiters, to the output string.
   21: COP(nibble[nib],MAC_String.DATA[index],2)MOV(46,MAC_String.DATA[index+2])ADD(nib,2,nib)ADD(index,3,index);
   22: COP(nibble[nib],MAC_String.DATA[index],2)MOV(46,MAC_String.DATA[index+2])ADD(nib,2,nib)ADD(index,3,index);
   23: COP(nibble[nib],MAC_String.DATA[index],2)MOV(46,MAC_String.DATA[index+2])ADD(nib,2,nib)ADD(index,3,index);
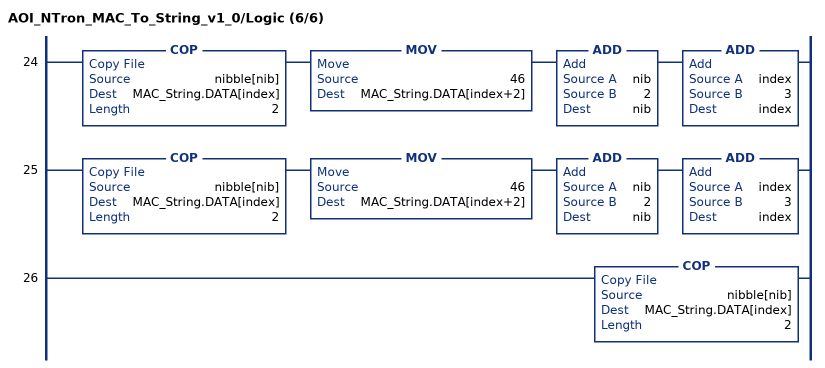
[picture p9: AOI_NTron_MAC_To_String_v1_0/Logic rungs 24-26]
   24: COP(nibble[nib],MAC_String.DATA[index],2)MOV(46,MAC_String.DATA[index+2])ADD(nib,2,nib)ADD(index,3,index);
   25: COP(nibble[nib],MAC_String.DATA[index],2)MOV(46,MAC_String.DATA[index+2])ADD(nib,2,nib)ADD(index,3,index);
   26: COP(nibble[nib],MAC_String.DATA[index],2);
END_ROUTINE
END_ADD_ON_INSTRUCTION

ADD_ON_INSTRUCTION AOI_NTron_String_Copy2_v1_0   (* revision 1.0, vendor Red Lion Controls, Inc. *)
// Copy a string formatted as a CIP STRING to an output STRING.
// (C) 2015 Red Lion Controls, Inc. All rights reserved.
VAR_IN_OUT
   Input_Length : INT; {required}
   Output : STRING; {required}
   Input_data : SINT; {required}
END_VAR
VAR
   size : DINT;
END_VAR

ROUTINE Logic   (* ladder *)
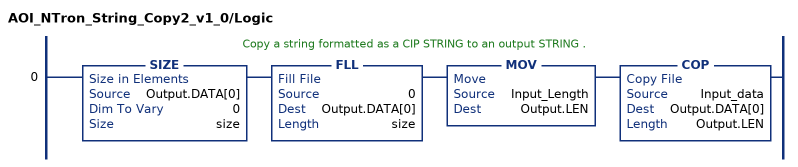
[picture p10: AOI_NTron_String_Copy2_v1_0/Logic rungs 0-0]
   // Copy a string formatted as a CIP STRING to an output STRING .
   0: SIZE(Output.DATA[0],0,size)FLL(0,Output.DATA[0],size)MOV(Input_Length,Output.LEN)COP(Input_data,Output.DATA[0],Output.LEN);
END_ROUTINE
END_ADD_ON_INSTRUCTION

ADD_ON_INSTRUCTION AOI_NTron_String_Copy_v1_0   (* revision 1.0, vendor Red Lion Controls, Inc. *)
// Copy a string formatted as a CIP SHORT_STRING to an output STRING.
// (C) 2015 Red Lion Controls, Inc. All rights reserved.
VAR_IN_OUT
   Input : SINT[100]; {required}
   Output : STRING; {required}
   indexInOut : DINT; {required}
END_VAR
VAR
   index : DINT;
END_VAR

ROUTINE Logic   (* ladder *)
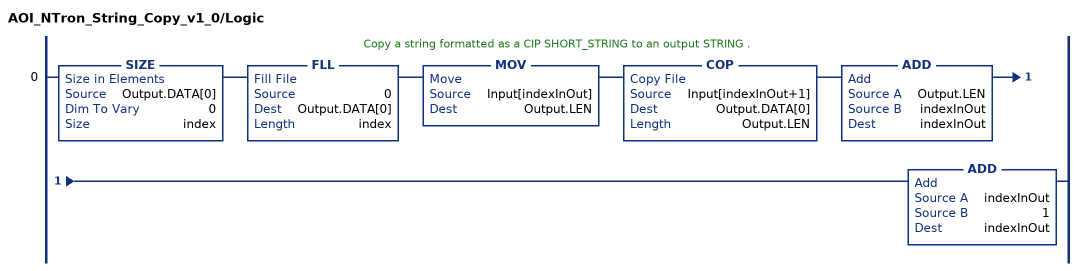
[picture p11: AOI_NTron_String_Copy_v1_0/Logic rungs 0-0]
   // Copy a string formatted as a CIP SHORT_STRING to an output STRING .
   0: SIZE(Output.DATA[0],0,index)FLL(0,Output.DATA[0],index)MOV(Input[indexInOut],Output.LEN)COP(Input[indexInOut+1],Output.DATA[0],Output.LEN)ADD(Output.LEN,indexInOut,indexInOut)ADD(indexInOut,1,indexInOut);
END_ROUTINE
END_ADD_ON_INSTRUCTION

ADD_ON_INSTRUCTION AOI_NTron_Sum_Port_Errors_v1_0   (* revision 1.0, vendor Red Lion Controls, Inc. *)
// Return an error count, and fault count, based on various port statistics.
// (C) 2015 Red Lion Controls, Inc. All rights reserved.
// Help:
// Error count is sum of single collisions, multiple collisions, late collisions, and deferred transmissions.
// Fault count is sum of alignment errors, FCS errors, SQE Test errors, excessive collisions, MAC transmit errors, carrier sense errors, frame too long, and MAC receive errors.
VAR_IN_OUT
   Ethernet_Link : UDT_NTRON_CIP_Ethernet_Link_v0; {required}
   Error_Count : DINT; {required}
   Fault_Count : DINT; {required}
END_VAR

ROUTINE Logic   (* ladder *)
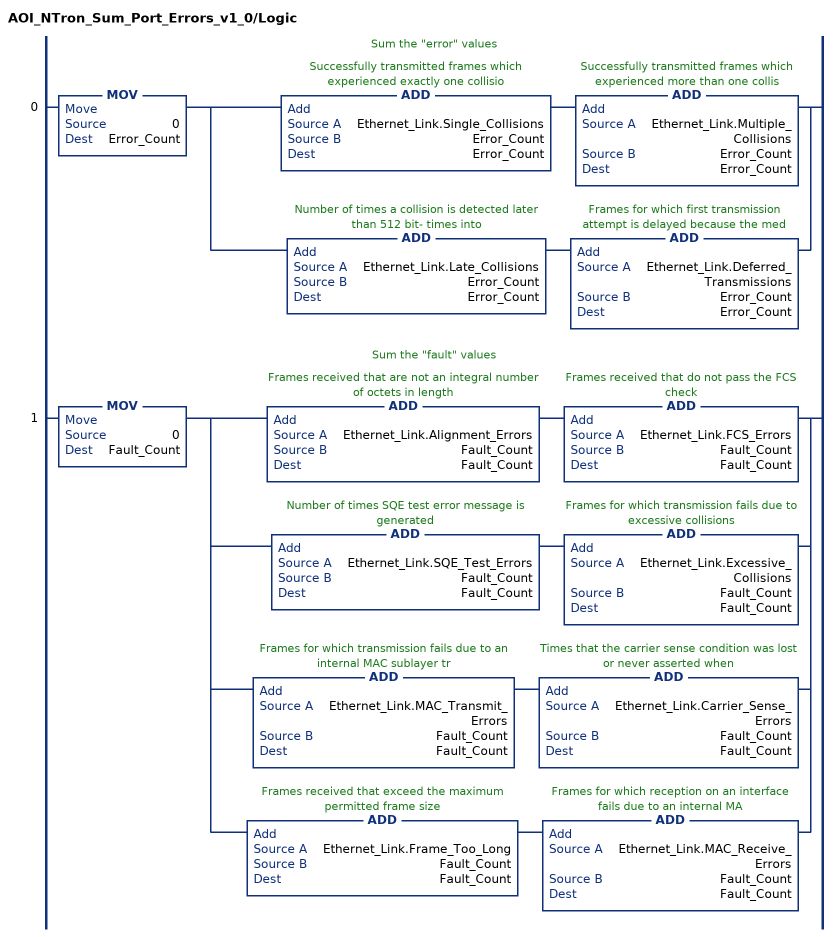
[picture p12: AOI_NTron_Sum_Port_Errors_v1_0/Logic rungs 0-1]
   // Sum the "error" values
   0: MOV(0,Error_Count)[ADD(Ethernet_Link.Single_Collisions,Error_Count,Error_Count) ADD(Ethernet_Link.Multiple_Collisions,Error_Count,Error_Count) ,ADD(Ethernet_Link.Late_Collisions,Error_Count,Error_Count) ADD(Ethernet_Link.Deferred_Transmissions,Error_Count,Error_Count) ];
   // Sum the "fault" values
   1: MOV(0,Fault_Count)[ADD(Ethernet_Link.Alignment_Errors,Fault_Count,Fault_Count) ADD(Ethernet_Link.FCS_Errors,Fault_Count,Fault_Count) ,ADD(Ethernet_Link.SQE_Test_Errors,Fault_Count,Fault_Count) ADD(Ethernet_Link.Excessive_Collisions,Fault_Count,Fault_Count) ,ADD(Ethernet_Link.MAC_Transmit_Errors,Fault_Count,Fault_Count) ADD(Ethernet_Link.Carrier_Sense_Errors,Fault_Count,Fault_Count) ,ADD(Ethernet_Link.Frame_Too_Long,Fault_Count,Fault_Count) ADD(Ethernet_Link.MAC_Receive_Errors,Fault_Count,Fault_Count) ];
END_ROUTINE
END_ADD_ON_INSTRUCTION

ADD_ON_INSTRUCTION AOI_NTron_Common_v1_2   (* revision 1.2 December 2015, vendor Red Lion Controls, Inc. *)
// Auxiliary AOI for N-Tron switches.
// (C) 2015 Red Lion Controls, Inc. All rights reserved.
// Overall version: 1.8
// Revision note:
// Overall Revision Notes
// 1.2 - Switch specific AOIs and other enhancements.
// 1.3.0 - Added AOIs for 711FX3, 7010TX, 709FX, 710FX2, 714FX6, and 712FX4 switches.
// 1.4.0 - June 2010. Added AOI for 7012FX2
// 1.5.0 - January 2011. Added AOI for 7026T
// 1.6.0 - February 2012. Added AOI for 7900
// 1.7.0 - August 2012. Added AOI for 716M12
// 1.8 - December 2015. Added support for CIP version 1.7
// Help:
// Refer to the installation document for more details.
// Revision 1.1 - changed messageCounter.PRE (preset) from 25 to 70. Initialize index and temp_int to 0.
VAR_IN_OUT
   Switch_Inputs : DINT[26]; {required}   // The module defined array representing the input assembly
        [5]   // Set utilization alarm flags for first 32 ports
   Switch_Output : DINT[1]; {required}   // The module defined array representing the output assembly
   Switch_Parameters : UDT_NTRON_Switch_Common_v1; {required}   // The primary AOI tag structure containing view of the input assembly and CIP object data
        .SWITCH.POWER_CONFIGURATION   // Power configuration
        .DATA.PORT_INTERFACE_TYPE   // Main operand description
END_VAR
VAR_OUTPUT
   Error : BOOL; {access Read Only}
END_VAR
VAR_IN_OUT
   Get_Message : MESSAGE; {required}   // Internal use: get all attributes
   Get_Message_Extended : MESSAGE; {required}   // Internal use: get all attributes, including vendor specific additions
   Storage : SINT[1200]; {required}   // Internal use: storage for explicit messaging responses
   Set_Message : MESSAGE; {required}   // Internal use: set single attribute
   SetData : INT[2]; {required}   // Internal use: data for set single attribute
END_VAR
VAR
   boolean : DINT;
   kRead_SwitchTrigger : SINT := 3;
   kRead_TCPIPTrigger : SINT := 2;
   kRead_IdentityTrigger : SINT := 1;
   kRead_PortTrigger : SINT := 4;
   kObjectClassEthernetLink : INT := 246;
   kObjectClassIdentity : INT := 1;
   kObjectClassTCPIP : INT := 245;   // k - first character - indicates a constant
   kObjectClassSwitch : INT := 192;
   messageCounter : COUNTER := (PRE := 50);
        .PRE   // The messageCounter preset must be at least 3 (Identity, TCPIP, and Switch objects) plus the maximum number of ports.
   messageTimer : TIMER := (PRE := 5000);
   bReadTCPIP : BOOL;
   bReadIdentity : BOOL;
   bReadSwitch : BOOL;
   bReadSwitchONS : BOOL;
   bReadIdentityONS : BOOL;
   bReadTCPIPONS : BOOL;
   bReadDoneONS : BOOL;
   bReadDone : BOOL;
   class : INT;
   temp_int : INT;
   oStringCopy2 : AOI_NTron_String_Copy2_v1_0;
   oIpAddressToString : AOI_NTron_IP_Address_to_String_v1_0;
   kServiceGetAllAttrExtended : SINT := 16#32;   // Get all attributes, including vendor specific additions
   nUpdateCounterEqualCount : INT;   // Counter incremented when update counter equals previous update counter
   port : INT;
   kMaxPortNumber : INT := 64;
   bReadPortONS : BOOL;
   bReadPort : BOOL;
   oStringCopy : AOI_NTron_String_Copy_v1_0;
   oIpAddressToString2 : AOI_NTron_IP_Address_to_String_v1_0;
   uptime : DINT;
   uptime_error : DINT;
   index : DINT;
   kAttributeAdminEnable : INT := 9;
   kAttributeSpeedDuplex : INT := 6;
   port_mask2 : DINT;
   port_mask : DINT;
   bReadExtendedDoneONS : BOOL;
   bReadExtendedDone : BOOL;
   bRequestData : BOOL;
   bResetCounter : BOOL;
   nStorageIndex : DINT;
   oStringCopy_2 : AOI_NTron_String_Copy_v1_0;
   oStringCopy_3 : AOI_NTron_String_Copy_v1_0;
   oMacToString : AOI_NTron_MAC_To_String_v1_0;
   MAC : SINT[6];
   nSize : INT;
   nUpdateCounter : INT;   // Saved value of assembly update counter
   bSetMessage : BOOL;
   oInterfaceControl : UDT_NTRON_CIP_Interface_Control_v0;
   nAdminSum : DINT;
   copyTimer : TIMER := (PRE := 5000);
   oSumPortErrors : AOI_NTron_Sum_Port_Errors_v1_0;
   kCIPMinorVersion : DINT;   // The AOI compares this version to the CIP Identity object version to determine if the AOI is compatible with the switch CIP version.
   kCIPMajorVersion : DINT;   // The AOI compares this version to the CIP Identity object version to determine if the AOI is compatible with the switch CIP version.
   bCIPVersionFault : BOOL;   // True if there is a CIP version fault
   oStringCopy3 : AOI_NTron_String_Copy_v1_0;
   oCIPStringICopy : AOI_NTron_CIP_STRINGI_Copy_v1_0;
   oStringICopy6 : AOI_NTron_CIP_STRINGI_Copy_v1_0;
   oStringICopy4 : AOI_NTron_CIP_STRINGI_Copy_v1_0;
END_VAR

ROUTINE Logic   (* ladder *)
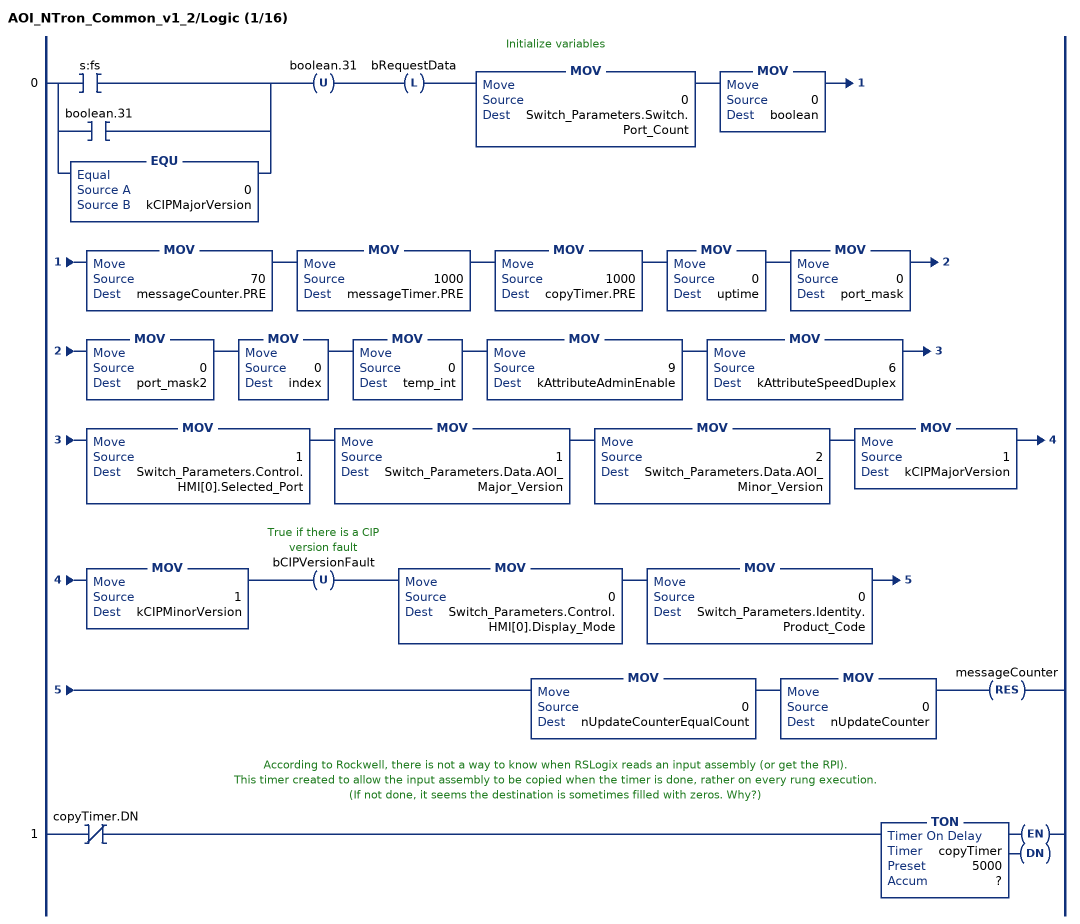
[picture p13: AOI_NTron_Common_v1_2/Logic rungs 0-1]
   // Initialize variables
   0: [XIC(s:fs) ,XIC(boolean.31) ,EQU(0,kCIPMajorVersion) ]OTU(boolean.31)OTL(bRequestData)MOV(0,Switch_Parameters.Switch.Port_Count)MOV(0,boolean)MOV(70,messageCounter.PRE)MOV(1000,messageTimer.PRE)MOV(1000,copyTimer.PRE)MOV(0,uptime)MOV(0,port_mask)MOV(0,port_mask2)MOV(0,index)MOV(0,temp_int)MOV(9,kAttributeAdminEnable)MOV(6,kAttributeSpeedDuplex)MOV(1,Switch_Parameters.Control.HMI[0].Selected_Port)MOV(1,Switch_Parameters.Data.AOI_Major_Version)MOV(2,Switch_Parameters.Data.AOI_Minor_Version)MOV(1,kCIPMajorVersion)MOV(1,kCIPMinorVersion)OTU(bCIPVersionFault)MOV(0,Switch_Parameters.Control.HMI[0].Display_Mode)MOV(0,Switch_Parameters.Identity.Product_Code)MOV(0,nUpdateCounterEqualCount)MOV(0,nUpdateCounter)RES(messageCounter);
   // According to Rockwell, there is not a way to know when RSLogix reads an input assembly (or get the RPI).
   // This timer created to allow the input assembly to be copied when the timer is done, rather on every rung execution.
   // (If not done, it seems the destination is sometimes filled with zeros. Why?)
   1: XIO(copyTimer.DN)TON(copyTimer,?,?);
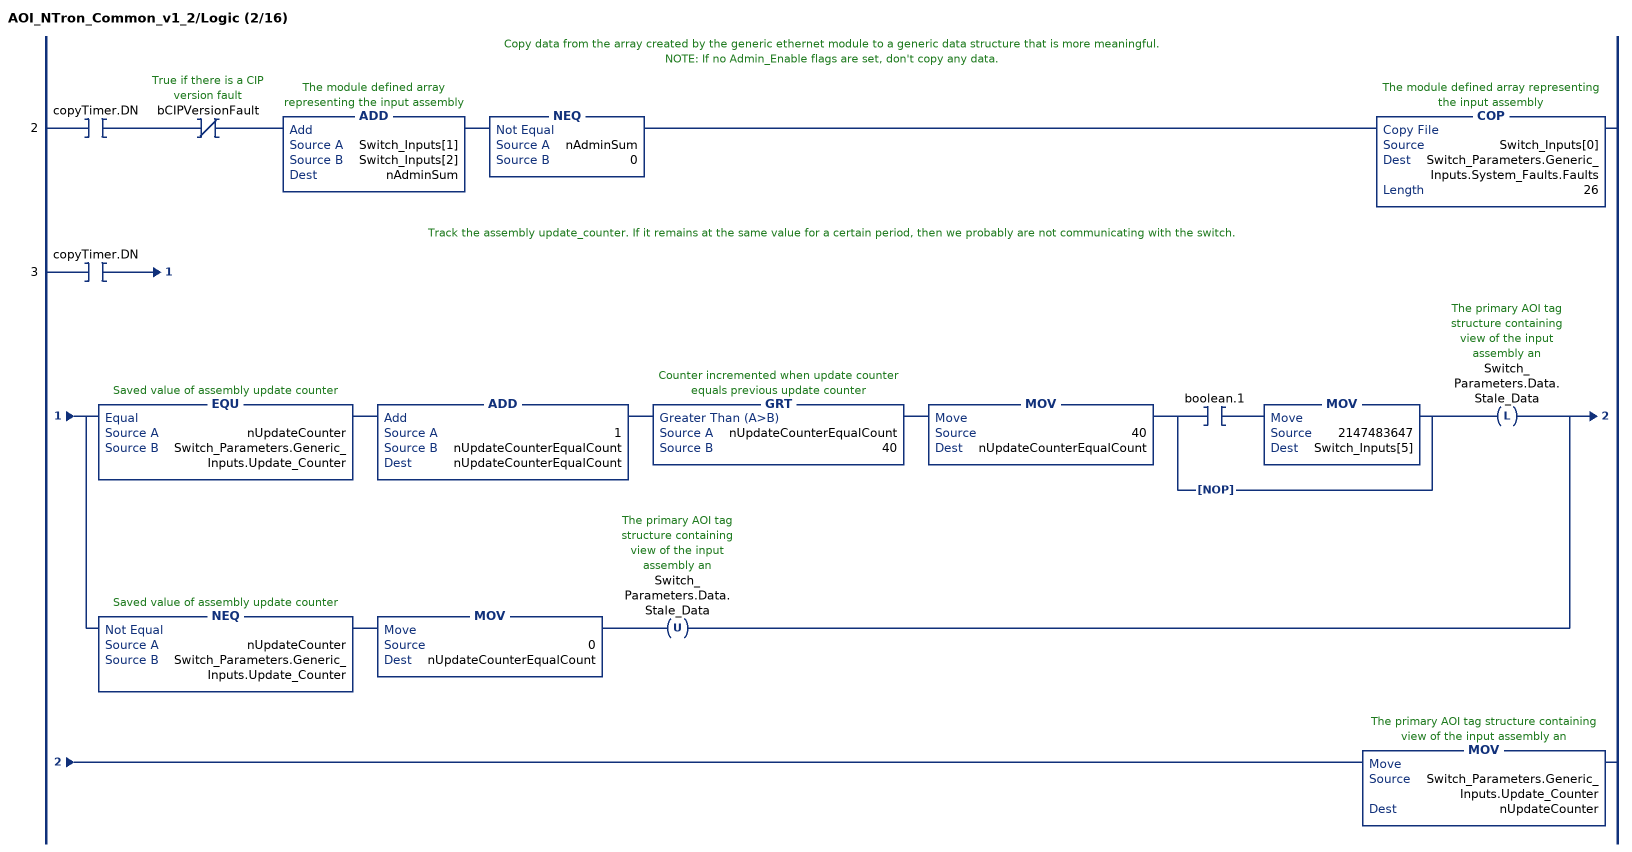
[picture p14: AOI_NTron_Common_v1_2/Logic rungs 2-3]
   // Copy data from the array created by the generic ethernet module to a generic data structure that is more meaningful.
   // NOTE: If no Admin_Enable flags are set, don't copy any data.
   2: XIC(copyTimer.DN)XIO(bCIPVersionFault)ADD(Switch_Inputs[1],Switch_Inputs[2],nAdminSum)NEQ(nAdminSum,0)COP(Switch_Inputs[0],Switch_Parameters.Generic_Inputs.System_Faults.Faults,26);
   // Track the assembly update_counter. If it remains at the same value for a certain period, then we probably are not communicating with the switch.
   3: XIC(copyTimer.DN)[EQU(nUpdateCounter,Switch_Parameters.Generic_Inputs.Update_Counter) ADD(1,nUpdateCounterEqualCount,nUpdateCounterEqualCount) GRT(nUpdateCounterEqualCount,40) MOV(40,nUpdateCounterEqualCount) [XIC(boolean.1) MOV(2147483647,Switch_Inputs[5]) ,NOP() ] OTL(Switch_Parameters.Data.Stale_Data) ,NEQ(nUpdateCounter,Switch_Parameters.Generic_Inputs.Update_Counter) MOV(0,nUpdateCounterEqualCount) OTU(Switch_Parameters.Data.Stale_Data) ]MOV(Switch_Parameters.Generic_Inputs.Update_Counter,nUpdateCounter);
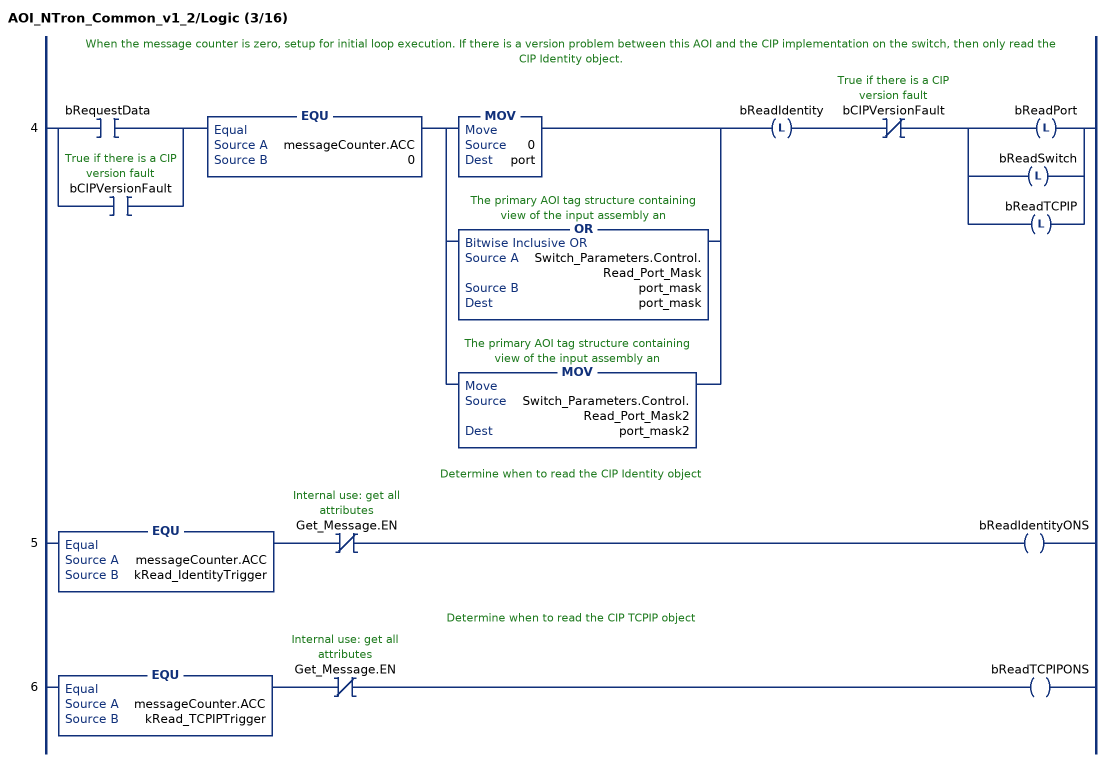
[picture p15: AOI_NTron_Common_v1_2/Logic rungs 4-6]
   // When the message counter is zero, setup for initial loop execution. If there is a version problem between this AOI and the CIP implementation on the switch, then only read the CIP Identity object.
   4: [XIC(bRequestData) ,XIC(bCIPVersionFault) ]EQU(messageCounter.ACC,0)[MOV(0,port) ,[OR(Switch_Parameters.Control.Read_Port_Mask,port_mask,port_mask) ,MOV(Switch_Parameters.Control.Read_Port_Mask2,port_mask2) ] ]OTL(bReadIdentity)XIO(bCIPVersionFault)[[OTL(bReadPort) ,OTL(bReadSwitch) ] ,OTL(bReadTCPIP) ];
   // Determine when to read the CIP Identity object
   5: EQU(messageCounter.ACC,kRead_IdentityTrigger)XIO(Get_Message.EN)OTE(bReadIdentityONS);
   // Determine when to read the CIP TCPIP object
   6: EQU(messageCounter.ACC,kRead_TCPIPTrigger)XIO(Get_Message.EN)OTE(bReadTCPIPONS);
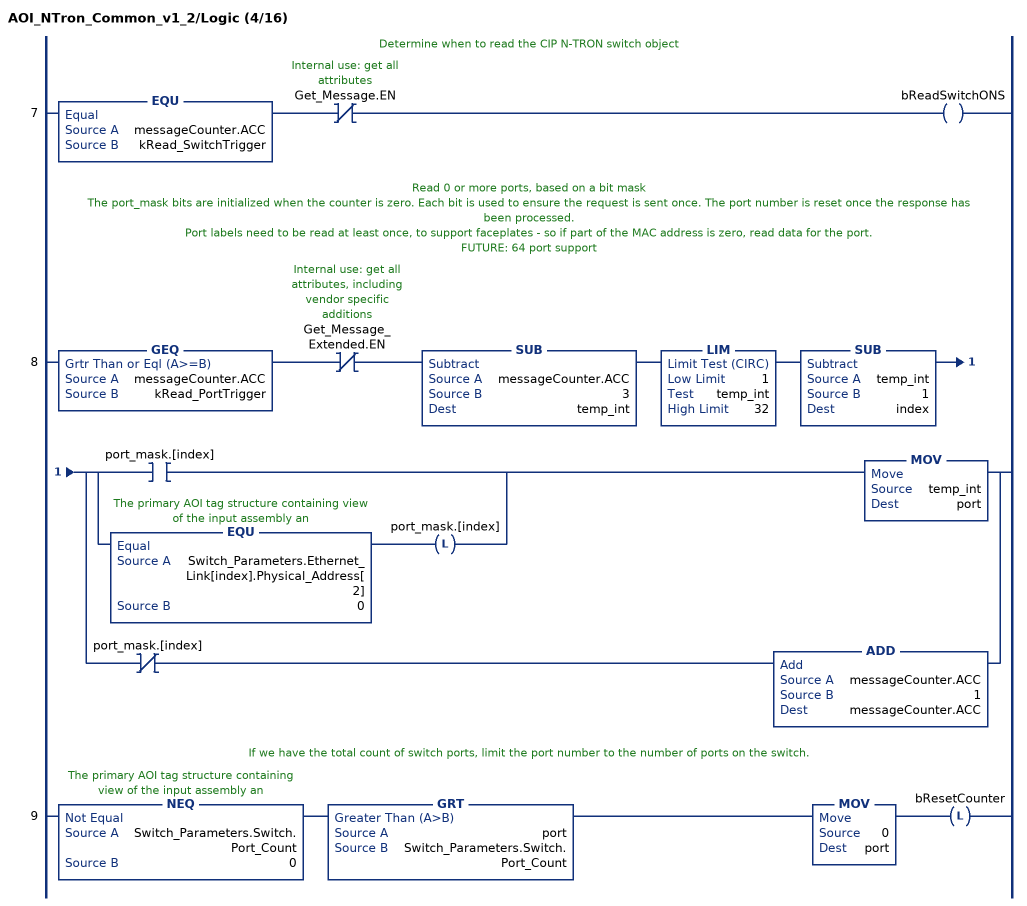
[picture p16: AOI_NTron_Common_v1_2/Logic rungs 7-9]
   // Determine when to read the CIP N-TRON switch object
   7: EQU(messageCounter.ACC,kRead_SwitchTrigger)XIO(Get_Message.EN)OTE(bReadSwitchONS);
   // Read 0 or more ports, based on a bit mask
   // The port_mask bits are initialized when the counter is zero. Each bit is used to ensure the request is sent once. The port number is reset once the response has been processed.
   // Port labels need to be read at least once, to support faceplates - so if part of the MAC address is zero, read data for the port.
   // FUTURE: 64 port support
   8: GEQ(messageCounter.ACC,kRead_PortTrigger)XIO(Get_Message_Extended.EN)SUB(messageCounter.ACC,3,temp_int)LIM(1,temp_int,32)SUB(temp_int,1,index)[[XIC(port_mask.[index]) ,EQU(Switch_Parameters.Ethernet_Link[index].Physical_Address[2],0) OTL(port_mask.[index]) ] MOV(temp_int,port) ,XIO(port_mask.[index]) ADD(messageCounter.ACC,1,messageCounter.ACC) ];
   // If we have the total count of switch ports, limit the port number to the number of ports on the switch.
   9: NEQ(Switch_Parameters.Switch.Port_Count,0)GRT(port,Switch_Parameters.Switch.Port_Count)MOV(0,port)OTL(bResetCounter);
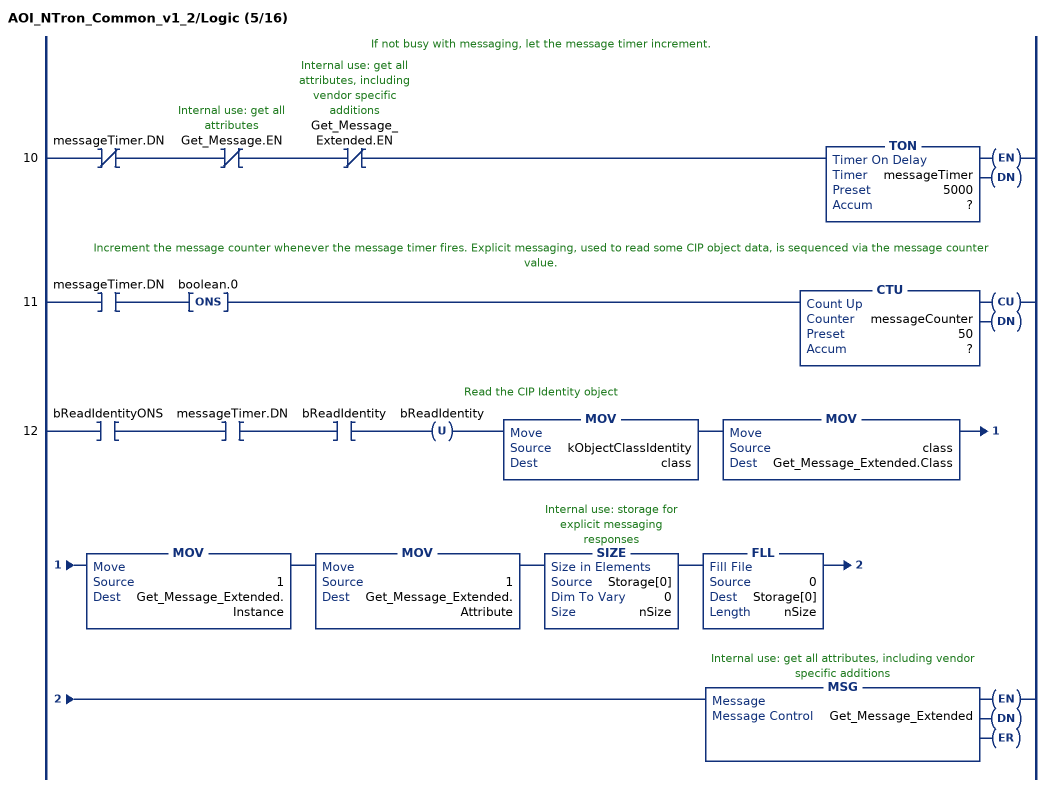
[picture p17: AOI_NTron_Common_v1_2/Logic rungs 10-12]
   // If not busy with messaging, let the message timer increment.
   10: XIO(messageTimer.DN)XIO(Get_Message.EN)XIO(Get_Message_Extended.EN)TON(messageTimer,?,?);
   // Increment the message counter whenever the message timer fires. Explicit messaging, used to read some CIP object data, is sequenced via the message counter value.
   11: XIC(messageTimer.DN)ONS(boolean.0)CTU(messageCounter,?,?);
   // Read the CIP Identity object
   12: XIC(bReadIdentityONS)XIC(messageTimer.DN)XIC(bReadIdentity)OTU(bReadIdentity)MOV(kObjectClassIdentity,class)MOV(class,Get_Message_Extended.Class)MOV(1,Get_Message_Extended.Instance)MOV(1,Get_Message_Extended.Attribute)SIZE(Storage[0],0,nSize)FLL(0,Storage[0],nSize)MSG(Get_Message_Extended);
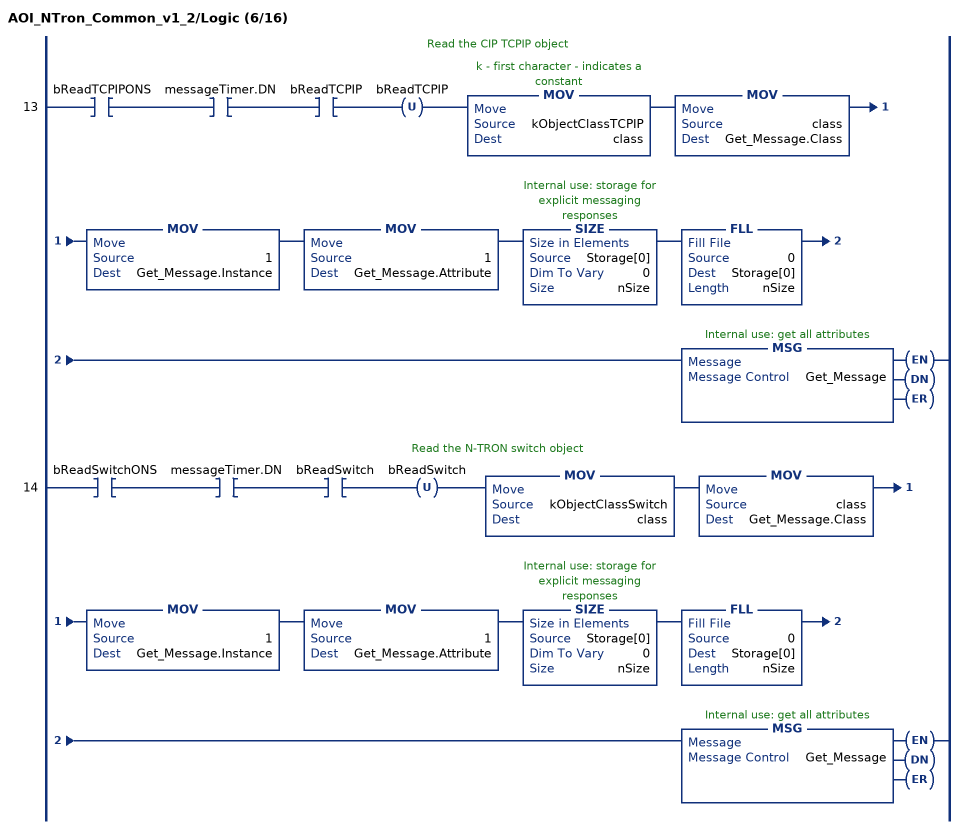
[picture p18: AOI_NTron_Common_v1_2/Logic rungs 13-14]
   // Read the CIP TCPIP object
   13: XIC(bReadTCPIPONS)XIC(messageTimer.DN)XIC(bReadTCPIP)OTU(bReadTCPIP)MOV(kObjectClassTCPIP,class)MOV(class,Get_Message.Class)MOV(1,Get_Message.Instance)MOV(1,Get_Message.Attribute)SIZE(Storage[0],0,nSize)FLL(0,Storage[0],nSize)MSG(Get_Message);
   // Read the N-TRON switch object
   14: XIC(bReadSwitchONS)XIC(messageTimer.DN)XIC(bReadSwitch)OTU(bReadSwitch)MOV(kObjectClassSwitch,class)MOV(class,Get_Message.Class)MOV(1,Get_Message.Instance)MOV(1,Get_Message.Attribute)SIZE(Storage[0],0,nSize)FLL(0,Storage[0],nSize)MSG(Get_Message);
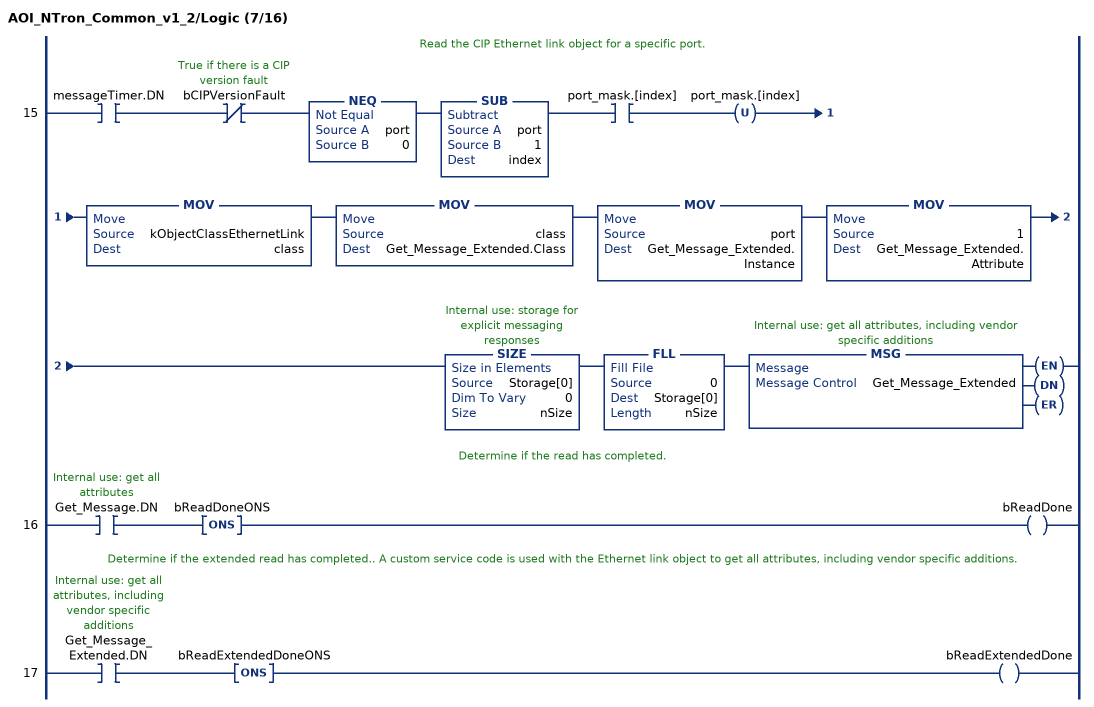
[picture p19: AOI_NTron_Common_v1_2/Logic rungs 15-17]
   // Read the CIP Ethernet link object for a specific port.
   15: XIC(messageTimer.DN)XIO(bCIPVersionFault)NEQ(port,0)SUB(port,1,index)XIC(port_mask.[index])OTU(port_mask.[index])MOV(kObjectClassEthernetLink,class)MOV(class,Get_Message_Extended.Class)MOV(port,Get_Message_Extended.Instance)MOV(1,Get_Message_Extended.Attribute)SIZE(Storage[0],0,nSize)FLL(0,Storage[0],nSize)MSG(Get_Message_Extended);
   // Determine if the read has completed.
   16: XIC(Get_Message.DN)ONS(bReadDoneONS)OTE(bReadDone);
   // Determine if the extended read has completed.. A custom service code is used with the Ethernet link object to get all attributes, including vendor specific additions.
   17: XIC(Get_Message_Extended.DN)ONS(bReadExtendedDoneONS)OTE(bReadExtendedDone);
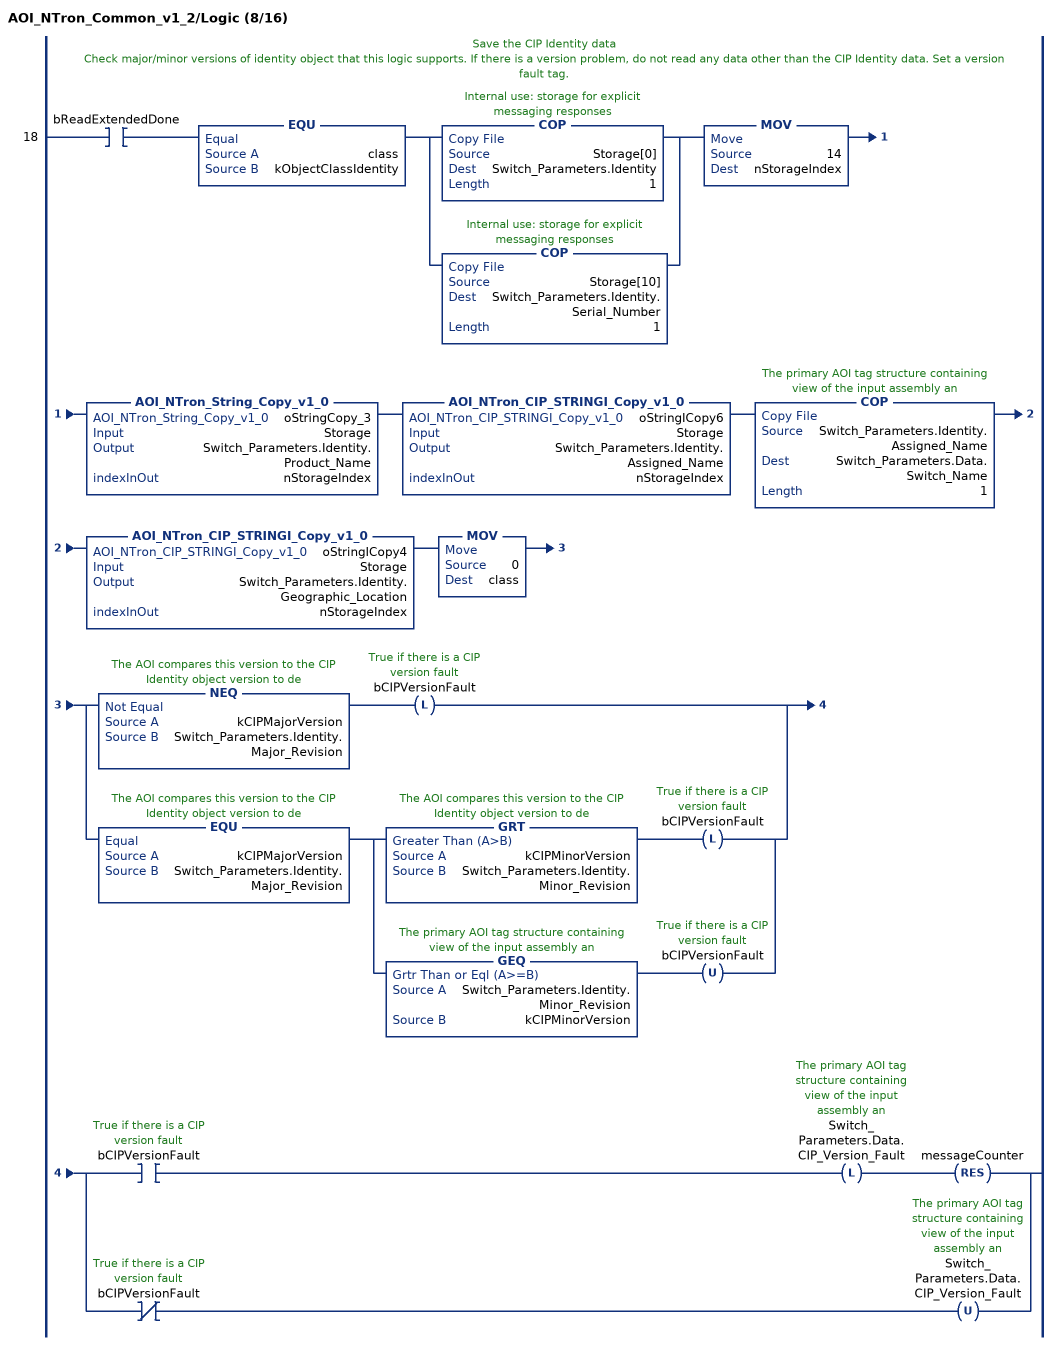
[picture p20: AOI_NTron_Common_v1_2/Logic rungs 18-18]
   // Save the CIP Identity data
   // Check major/minor versions of identity object that this logic supports. If there is a version problem, do not read any data other than the CIP Identity data. Set a version fault tag.
   18: XIC(bReadExtendedDone)EQU(class,kObjectClassIdentity)[COP(Storage[0],Switch_Parameters.Identity,1) ,COP(Storage[10],Switch_Parameters.Identity.Serial_Number,1) ]MOV(14,nStorageIndex)AOI_NTron_String_Copy_v1_0(oStringCopy_3,Storage,Switch_Parameters.Identity.Product_Name,nStorageIndex)AOI_NTron_CIP_STRINGI_Copy_v1_0(oStringICopy6,Storage,Switch_Parameters.Identity.Assigned_Name,nStorageIndex)COP(Switch_Parameters.Identity.Assigned_Name,Switch_Parameters.Data.Switch_Name,1)AOI_NTron_CIP_STRINGI_Copy_v1_0(oStringICopy4,Storage,Switch_Parameters.Identity.Geographic_Location,nStorageIndex)MOV(0,class)[NEQ(kCIPMajorVersion,Switch_Parameters.Identity.Major_Revision) OTL(bCIPVersionFault) ,EQU(kCIPMajorVersion,Switch_Parameters.Identity.Major_Revision) [GRT(kCIPMinorVersion,Switch_Parameters.Identity.Minor_Revision) OTL(bCIPVersionFault) ,GEQ(Switch_Parameters.Identity.Minor_Revision,kCIPMinorVersion) OTU(bCIPVersionFault) ] ][XIC(bCIPVersionFault) OTL(Switch_Parameters.Data.CIP_Version_Fault) RES(messageCounter) ,XIO(bCIPVersionFault) OTU(Switch_Parameters.Data.CIP_Version_Fault) ];
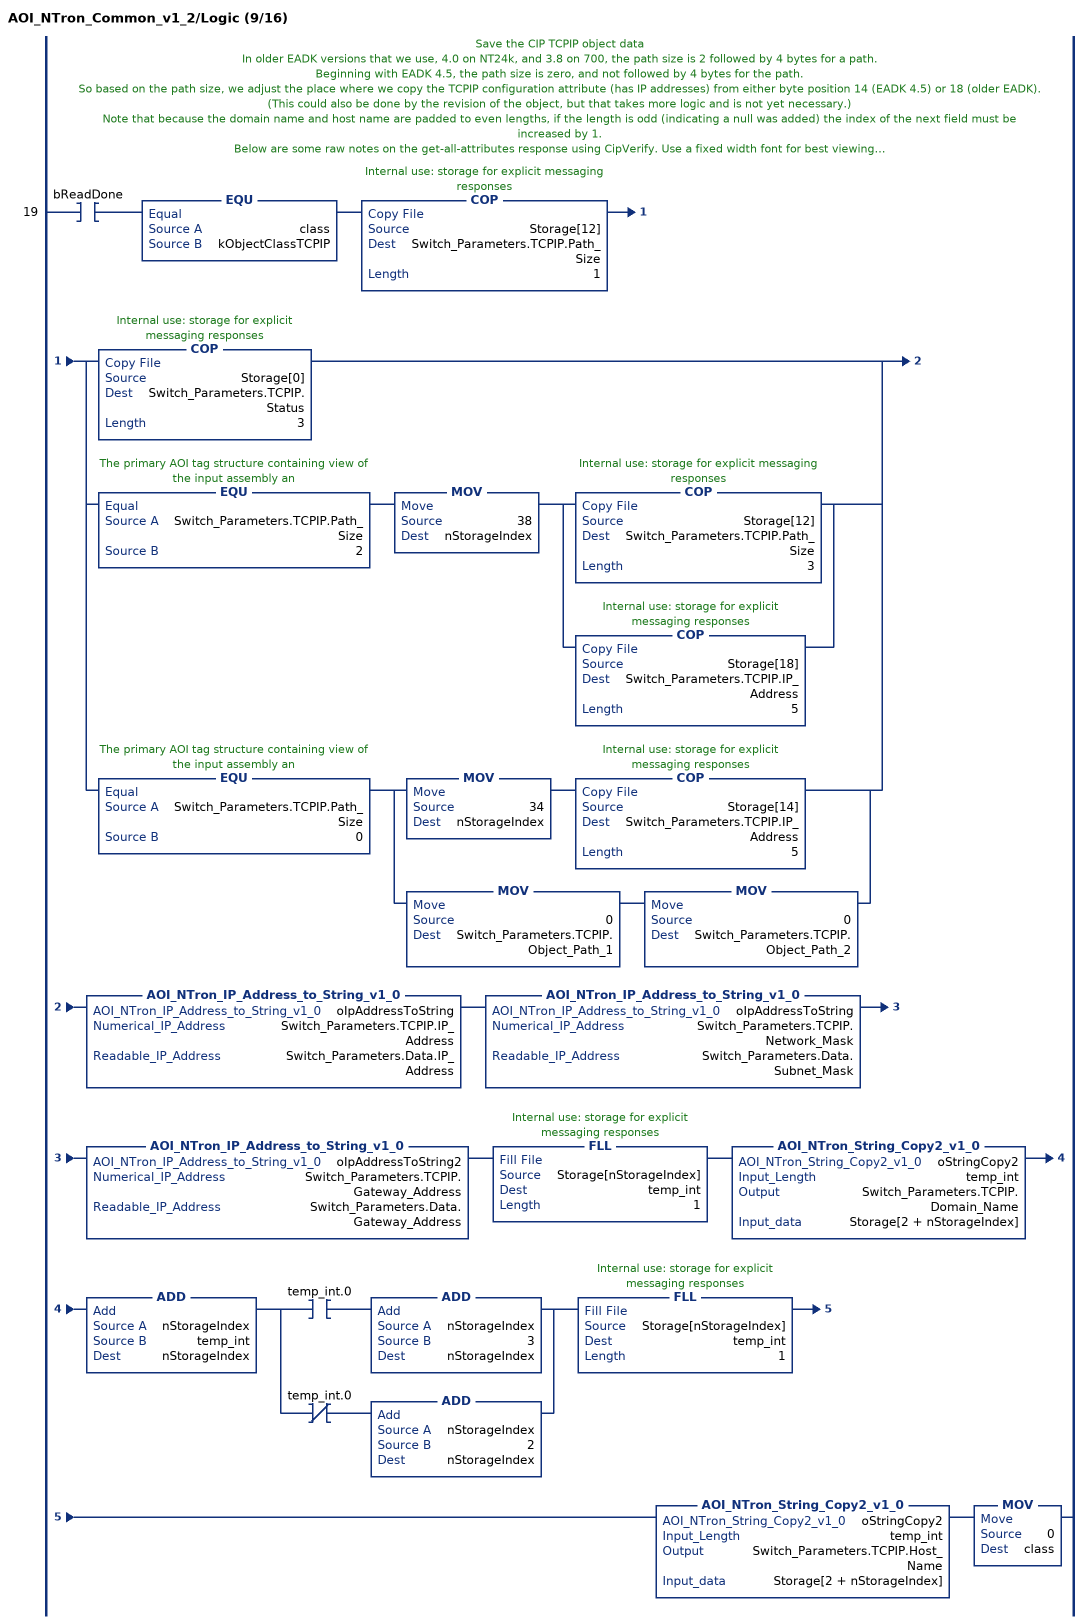
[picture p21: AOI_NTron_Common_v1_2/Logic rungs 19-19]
   // Save the CIP TCPIP object data
   // In older EADK versions that we use, 4.0 on NT24k, and 3.8 on 700, the path size is 2 followed by 4 bytes for a path.
   // Beginning with EADK 4.5, the path size is zero, and not followed by 4 bytes for the path.
   // So based on the path size, we adjust the place where we copy the TCPIP configuration attribute (has IP addresses) from either byte position 14 (EADK 4.5) or 18 (older EADK).
   // (This could also be done by the revision of the object, but that takes more logic and is not yet necessary.)
   // Note that because the domain name and host name are padded to even lengths, if the length is odd (indicating a null was added) the index of the next field must be increased by 1.
   // Below are some raw notes on the get-all-attributes response using CipVerify. Use a fixed width font for best viewing.
   // (ps-packet size, ip-IP address, sn-subnet mask, gw-gateway address, d1-domain server 1, d2- domain server 2, dn-domain name, hn-host name)
   //                                                                    ps                ip          sn          gw          d1          d2          dn    hn
   // [38]|GetAll, TCPIP, instance 1|01 00 00 00 14 00 00 00 00 00 00 00 02 00 20 F6 24 01 FB 14 10 AC 00 FF FF FF 01 14 10 AC 00 00 00 00 00 00 00 00 00 00 00 00
   //                                0  1  2  3  4  5  6  7  8  9  10 11 12 13 14 15 16 17 18 19 20 21 22 23 24 25 26 27 28 29 30 31 32 33 34 36 36 37 38 39 40 41
   //                                                                    ps    ip          sn          gw          d1          d2          dn    hn
   // [40]|GetAll, TCPIP, instance 1|01 00 00 00 54 00 00 00 00 00 00 00 00 00 FC 14 10 AC 00 FF FF FF 01 14 10 AC 00 00 00 00 00 00 00 00 00 00 00 00 00 00 00 00 00 00 01 00 00 01 00 60 20 C0 EF 00 00 00 00 00 00 00 00 00 00 00 00 00 00 00 00 00 00 00 00 00 00 00 00 00 00 00 00 00 00 00 00 00 00 00 00 00 78 00
   //                                0  1  2  3  4  5  6  7  8  9  10 11 12 13 14 15 16 17 18 19 20 21 22 23 24 25 26 27 28 29 30 31 32 33 34 36 36 37 38 39 40 41
   19: XIC(bReadDone)EQU(class,kObjectClassTCPIP)COP(Storage[12],Switch_Parameters.TCPIP.Path_Size,1)[COP(Storage[0],Switch_Parameters.TCPIP.Status,3) ,[EQU(Switch_Parameters.TCPIP.Path_Size,2) MOV(38,nStorageIndex) [COP(Storage[12],Switch_Parameters.TCPIP.Path_Size,3) ,COP(Storage[18],Switch_Parameters.TCPIP.IP_Address,5) ] ,EQU(Switch_Parameters.TCPIP.Path_Size,0) [MOV(34,nStorageIndex) COP(Storage[14],Switch_Parameters.TCPIP.IP_Address,5) ,MOV(0,Switch_Parameters.TCPIP.Object_Path_1) MOV(0,Switch_Parameters.TCPIP.Object_Path_2) ] ] ]AOI_NTron_IP_Address_to_String_v1_0(oIpAddressToString,Switch_Parameters.TCPIP.IP_Address,Switch_Parameters.Data.IP_Address)AOI_NTron_IP_Address_to_String_v1_0(oIpAddressToString,Switch_Parameters.TCPIP.Network_Mask,Switch_Parameters.Data.Subnet_Mask)AOI_NTron_IP_Address_to_String_v1_0(oIpAddressToString2,Switch_Parameters.TCPIP.Gateway_Address,Switch_Parameters.Data.Gateway_Address)FLL(Storage[nStorageIndex],temp_int,1)AOI_NTron_String_Copy2_v1_0(oStringCopy2,temp_int,Switch_Parameters.TCPIP.Domain_Name,Storage[2 + nStorageIndex])ADD(nStorageIndex,temp_int,nStorageIndex)[XIC(temp_int.0) ADD(nStorageIndex,3,nStorageIndex) ,XIO(temp_int.0) ADD(nStorageIndex,2,nStorageIndex) ]FLL(Storage[nStorageIndex],temp_int,1)AOI_NTron_String_Copy2_v1_0(oStringCopy2,temp_int,Switch_Parameters.TCPIP.Host_Name,Storage[2 + nStorageIndex])MOV(0,class);
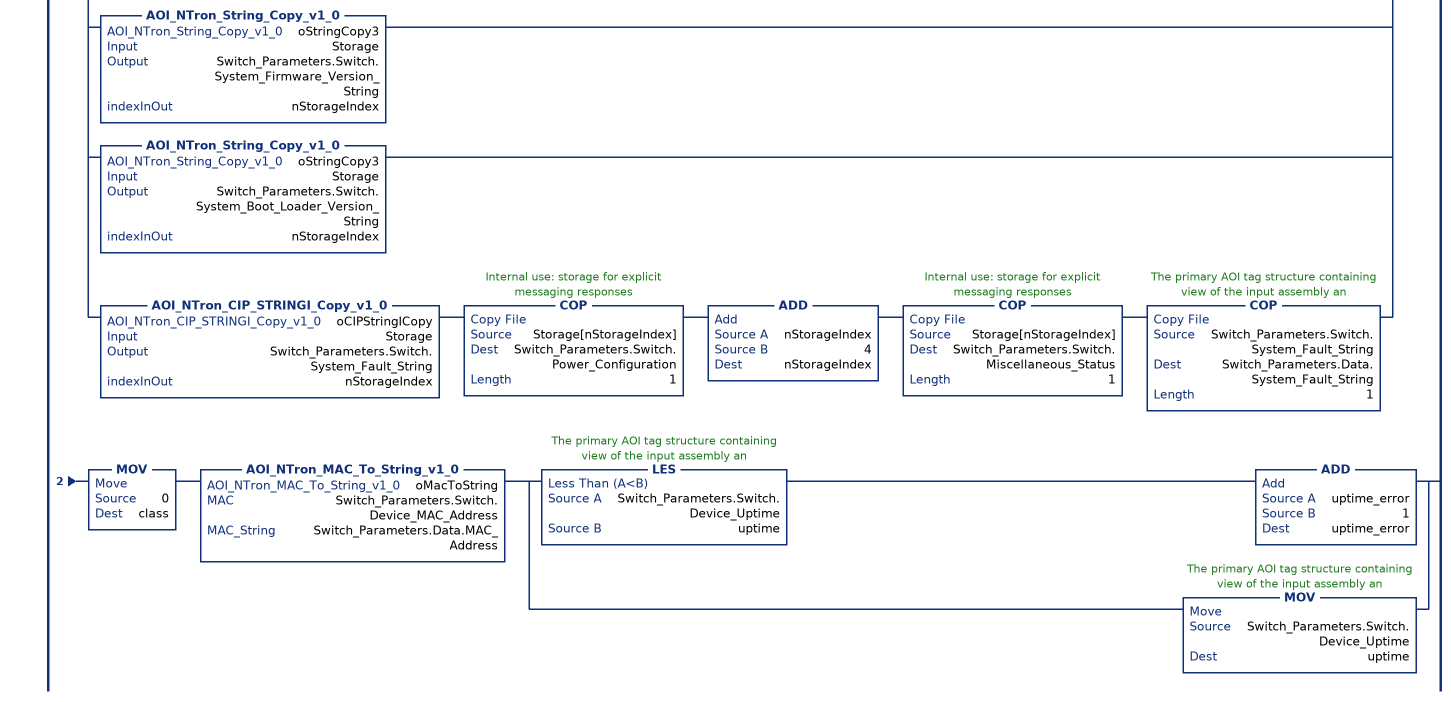
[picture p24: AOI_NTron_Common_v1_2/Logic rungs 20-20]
   // Save the CIP N-TRON switch object data.
   20: XIC(bReadDone)EQU(class,kObjectClassSwitch)MOV(0,nStorageIndex)[COP(Storage[nStorageIndex],Switch_Parameters.Switch.Device_Uptime,2) ADD(nStorageIndex,8,nStorageIndex) ,COP(Storage[nStorageIndex],Switch_Parameters.Switch.Valid_Ports[0],6) ADD(nStorageIndex,24,nStorageIndex) ,COP(Storage[nStorageIndex],Switch_Parameters.Switch.System_Faults,1) ADD(nStorageIndex,4,nStorageIndex) ,COP(Storage[nStorageIndex],Switch_Parameters.Switch.IGMP_Querier_Status,3) ADD(nStorageIndex,3,nStorageIndex) ,COP(Storage[nStorageIndex],Switch_Parameters.Switch.IGMP_Active_Querier,1) ADD(nStorageIndex,4,nStorageIndex) ,COP(Storage[nStorageIndex],Switch_Parameters.Switch.CPU_Usage,1) ADD(nStorageIndex,1,nStorageIndex) ,COP(Storage[nStorageIndex],Switch_Parameters.Switch.Class1_Connections,4) ADD(nStorageIndex,8,nStorageIndex) ,COP(Storage[nStorageIndex],Switch_Parameters.Switch.Contact_Status,1) ADD(nStorageIndex,1,nStorageIndex) ,COP(Storage[nStorageIndex],Switch_Parameters.Switch.Temperature_C,2) ADD(nStorageIndex,4,nStorageIndex) ,ADD(nStorageIndex,8,nStorageIndex) ,COP(Storage[nStorageIndex],Switch_Parameters.Switch.Device_MAC_Address[0],6) ADD(nStorageIndex,6,nStorageIndex) ,COP(Storage[nStorageIndex],Switch_Parameters.Switch.Device_Role,1) ADD(nStorageIndex,4,nStorageIndex) ,COP(Storage[nStorageIndex],Switch_Parameters.Switch.Config_Device_Status,1) ADD(nStorageIndex,1,nStorageIndex) ,COP(Storage[nStorageIndex],Switch_Parameters.Switch.System_Configuration,1) ADD(nStorageIndex,4,nStorageIndex) ,AOI_NTron_String_Copy_v1_0(oStringCopy3,Storage,Switch_Parameters.Switch.System_Firmware_Version_String,nStorageIndex) ,AOI_NTron_String_Copy_v1_0(oStringCopy3,Storage,Switch_Parameters.Switch.System_Boot_Loader_Version_String,nStorageIndex) ,AOI_NTron_CIP_STRINGI_Copy_v1_0(oCIPStringICopy,Storage,Switch_Parameters.Switch.System_Fault_String,nStorageIndex) COP(Storage[nStorageIndex],Switch_Parameters.Switch.Power_Configuration,1) ADD(nStorageIndex,4,nStorageIndex) COP(Storage[nStorageIndex],Switch_Parameters.Switch.Miscellaneous_Status,1) COP(Switch_Parameters.Switch.System_Fault_String,Switch_Parameters.Data.System_Fault_String,1) ]MOV(0,class)AOI_NTron_MAC_To_String_v1_0(oMacToString,Switch_Parameters.Switch.Device_MAC_Address,Switch_Parameters.Data.MAC_Address)[LES(Switch_Parameters.Switch.Device_Uptime,uptime) ADD(uptime_error,1,uptime_error) ,MOV(Switch_Parameters.Switch.Device_Uptime,uptime) ];
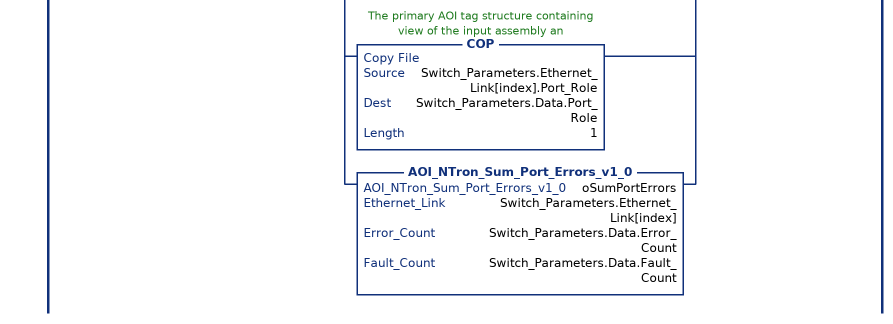
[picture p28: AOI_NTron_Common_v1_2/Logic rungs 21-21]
   // Save the CIP Ethernet link object data for a port
   21: XIC(bReadExtendedDone)EQU(class,kObjectClassEthernetLink)NEQ(port,0)SUB(port,1,index)[[COP(Storage[0],Switch_Parameters.Ethernet_Link[index].Interface_Speed,1) ,COP(Storage[4],Switch_Parameters.Ethernet_Link[index].Interface_Flags,1) ] ,[COP(Storage[8],Switch_Parameters.Ethernet_Link[index].Physical_Address[0],6) ,[COP(Storage[14],Switch_Parameters.Ethernet_Link[index].InOctets,23) ,[[COP(Storage[106],Switch_Parameters.Ethernet_Link[index].Control_Bits,2) ,COP(Storage[110],Switch_Parameters.Ethernet_Link[index].Interface_Type,3) ] ,MOV(113,nStorageIndex) AOI_NTron_String_Copy_v1_0(oStringCopy,Storage,Switch_Parameters.Ethernet_Link[index].Interface_Label,nStorageIndex) ,AOI_NTron_String_Copy_v1_0(oStringCopy_2,Storage,Switch_Parameters.Ethernet_Link[index].Interface_Description,nStorageIndex) ,COP(Storage[nStorageIndex],Switch_Parameters.Ethernet_Link[index].Interface_Utilization,4) ADD(nStorageIndex,4,nStorageIndex) ,COP(Storage[nStorageIndex],Switch_Parameters.Ethernet_Link[index].TX_Unicast_Packet_Rate,11) ADD(nStorageIndex,44,nStorageIndex) ] ] ] ]EQU(Switch_Parameters.Control.HMI[0].Selected_Port,port)MOV(port,Switch_Parameters.Data.Port)[COP(Switch_Parameters.Ethernet_Link[index].Interface_Flags,Switch_Parameters.Data.Port_Interface_Flags,1) ,COP(Switch_Parameters.Ethernet_Link[index].Interface_Speed,Switch_Parameters.Data.Port_Speed,1) ,COP(Switch_Parameters.Ethernet_Link[index].Interface_Type,Switch_Parameters.Data.Port_Interface_Type,1) ,COP(Switch_Parameters.Ethernet_Link[index].Interface_Label,Switch_Parameters.Data.Port_Interface_Label,1) ,COP(Switch_Parameters.Ethernet_Link[index].Interface_Utilization,Switch_Parameters.Data.Interface_Utilization,1) ,COP(Switch_Parameters.Ethernet_Link[index].InOctets,Switch_Parameters.Data.InOctets,3) ,COP(Switch_Parameters.Ethernet_Link[index].OutOctets,Switch_Parameters.Data.OutOctets,3) ,COP(Switch_Parameters.Ethernet_Link[index].TX_Unicast_Packet_Rate,Switch_Parameters.Data.TX_Unicast_Packet_Rate,6) ,COP(Switch_Parameters.Ethernet_Link[index].Physical_Address[0],MAC[0],6) ,COP(Switch_Parameters.Ethernet_Link[index].Port_Role,Switch_Parameters.Data.Port_Role,1) ,AOI_NTron_Sum_Port_Errors_v1_0(oSumPortErrors,Switch_Parameters.Ethernet_Link[index],Switch_Parameters.Data.Error_Count,Switch_Parameters.Data.Fault_Count) ][MOV(0,port) ,MOV(0,class) ];
